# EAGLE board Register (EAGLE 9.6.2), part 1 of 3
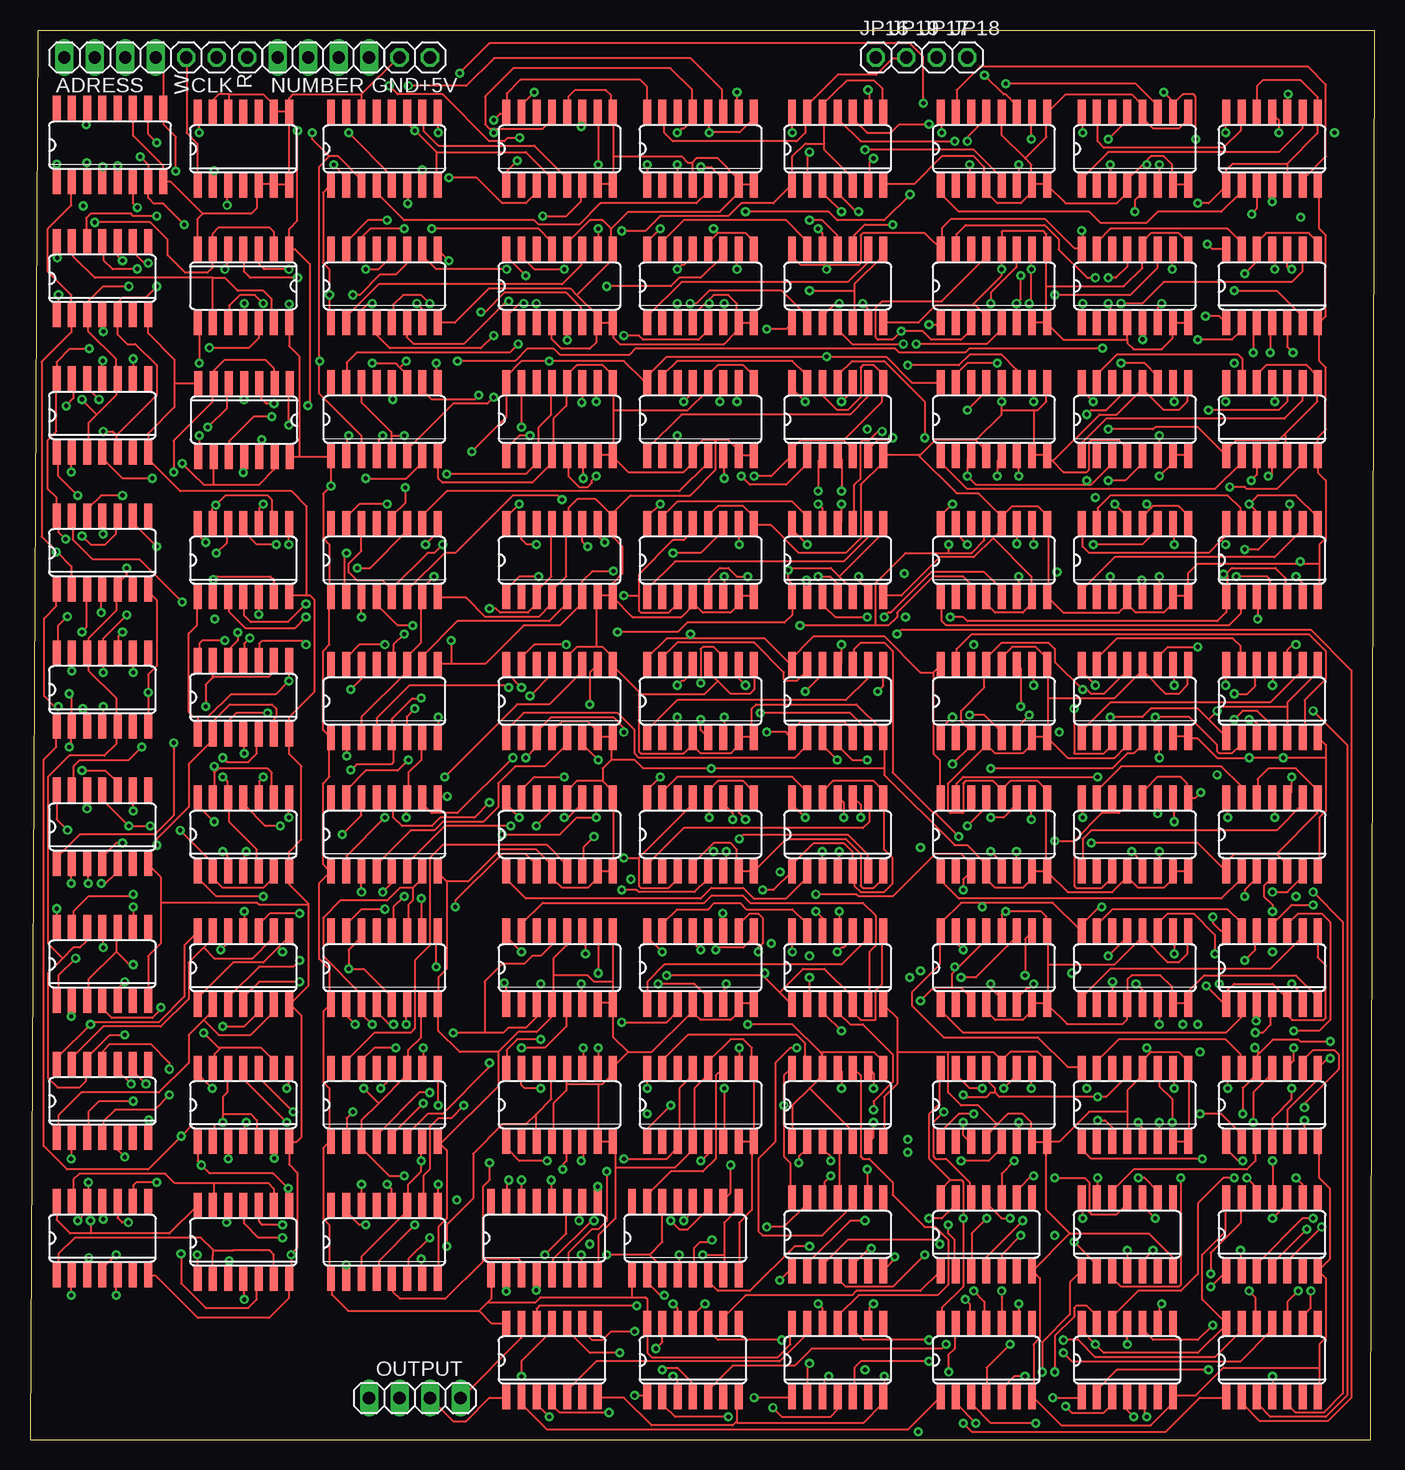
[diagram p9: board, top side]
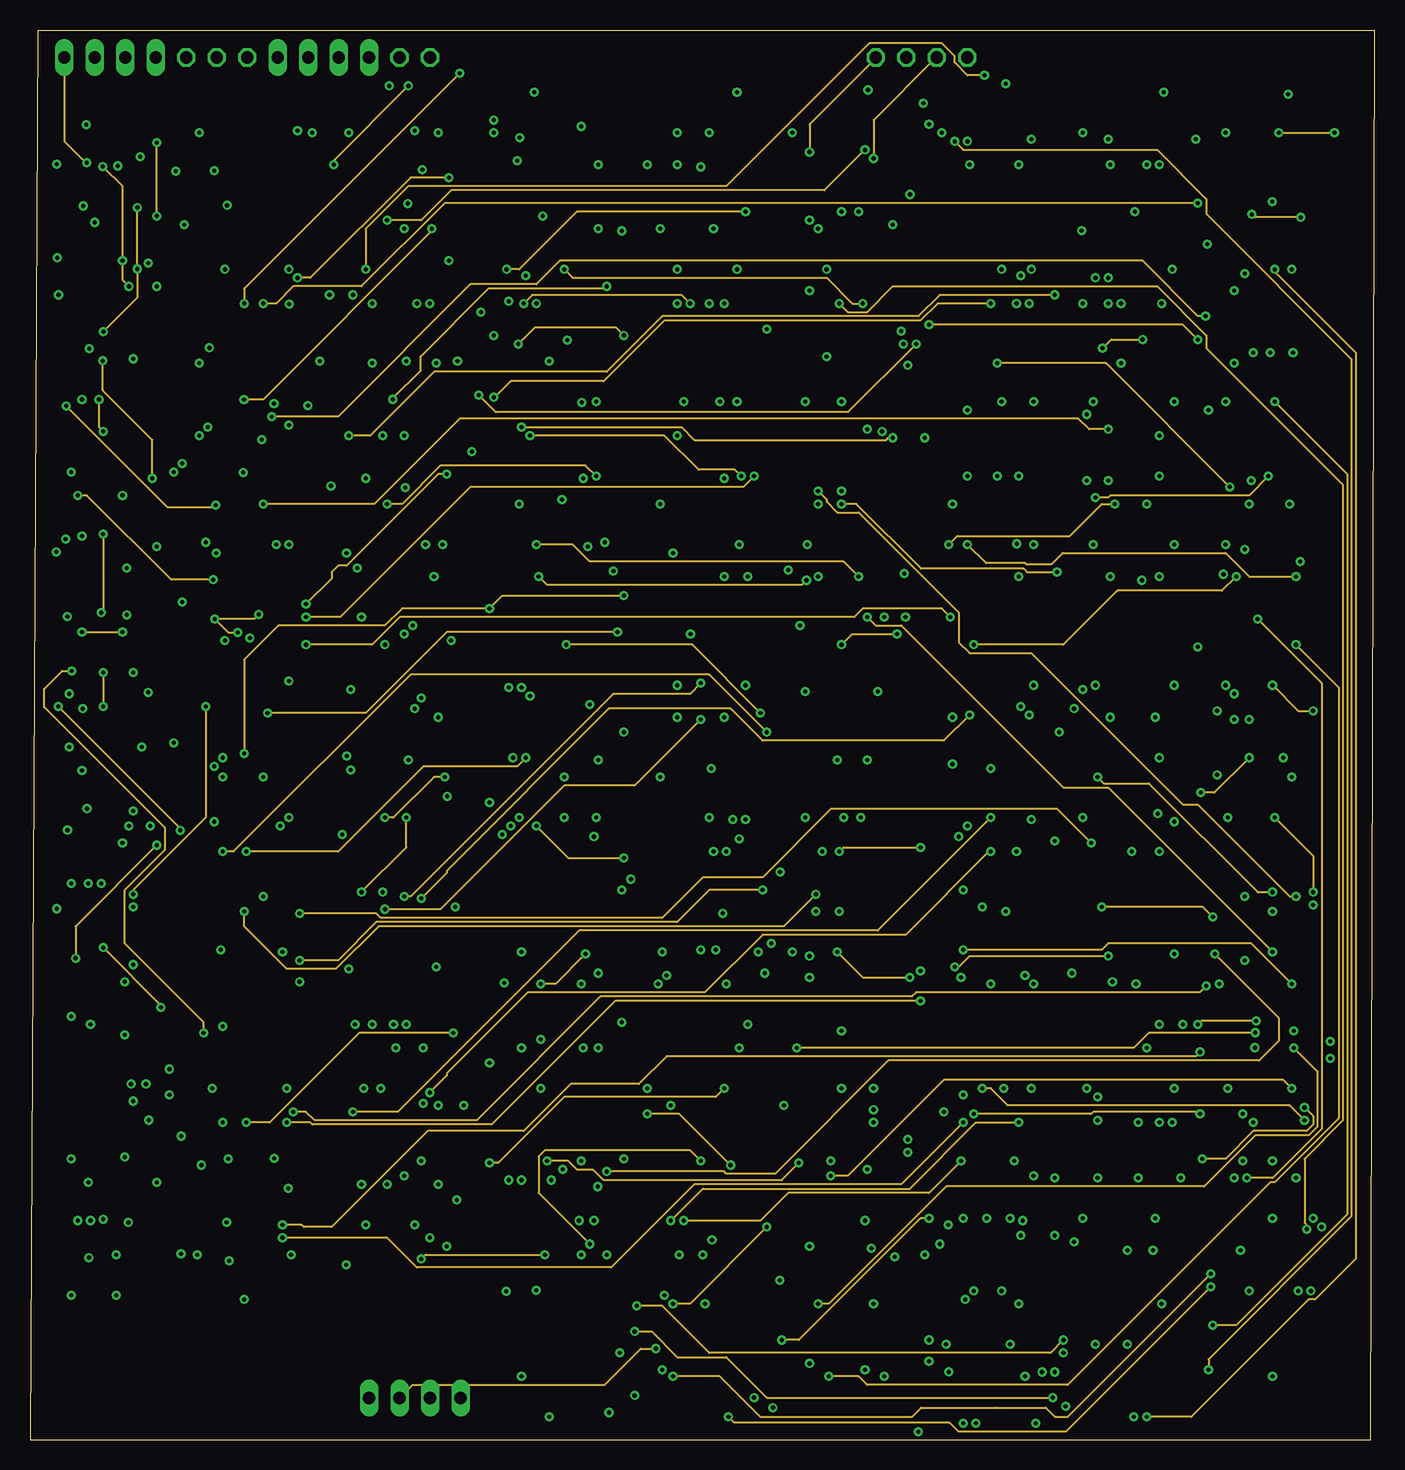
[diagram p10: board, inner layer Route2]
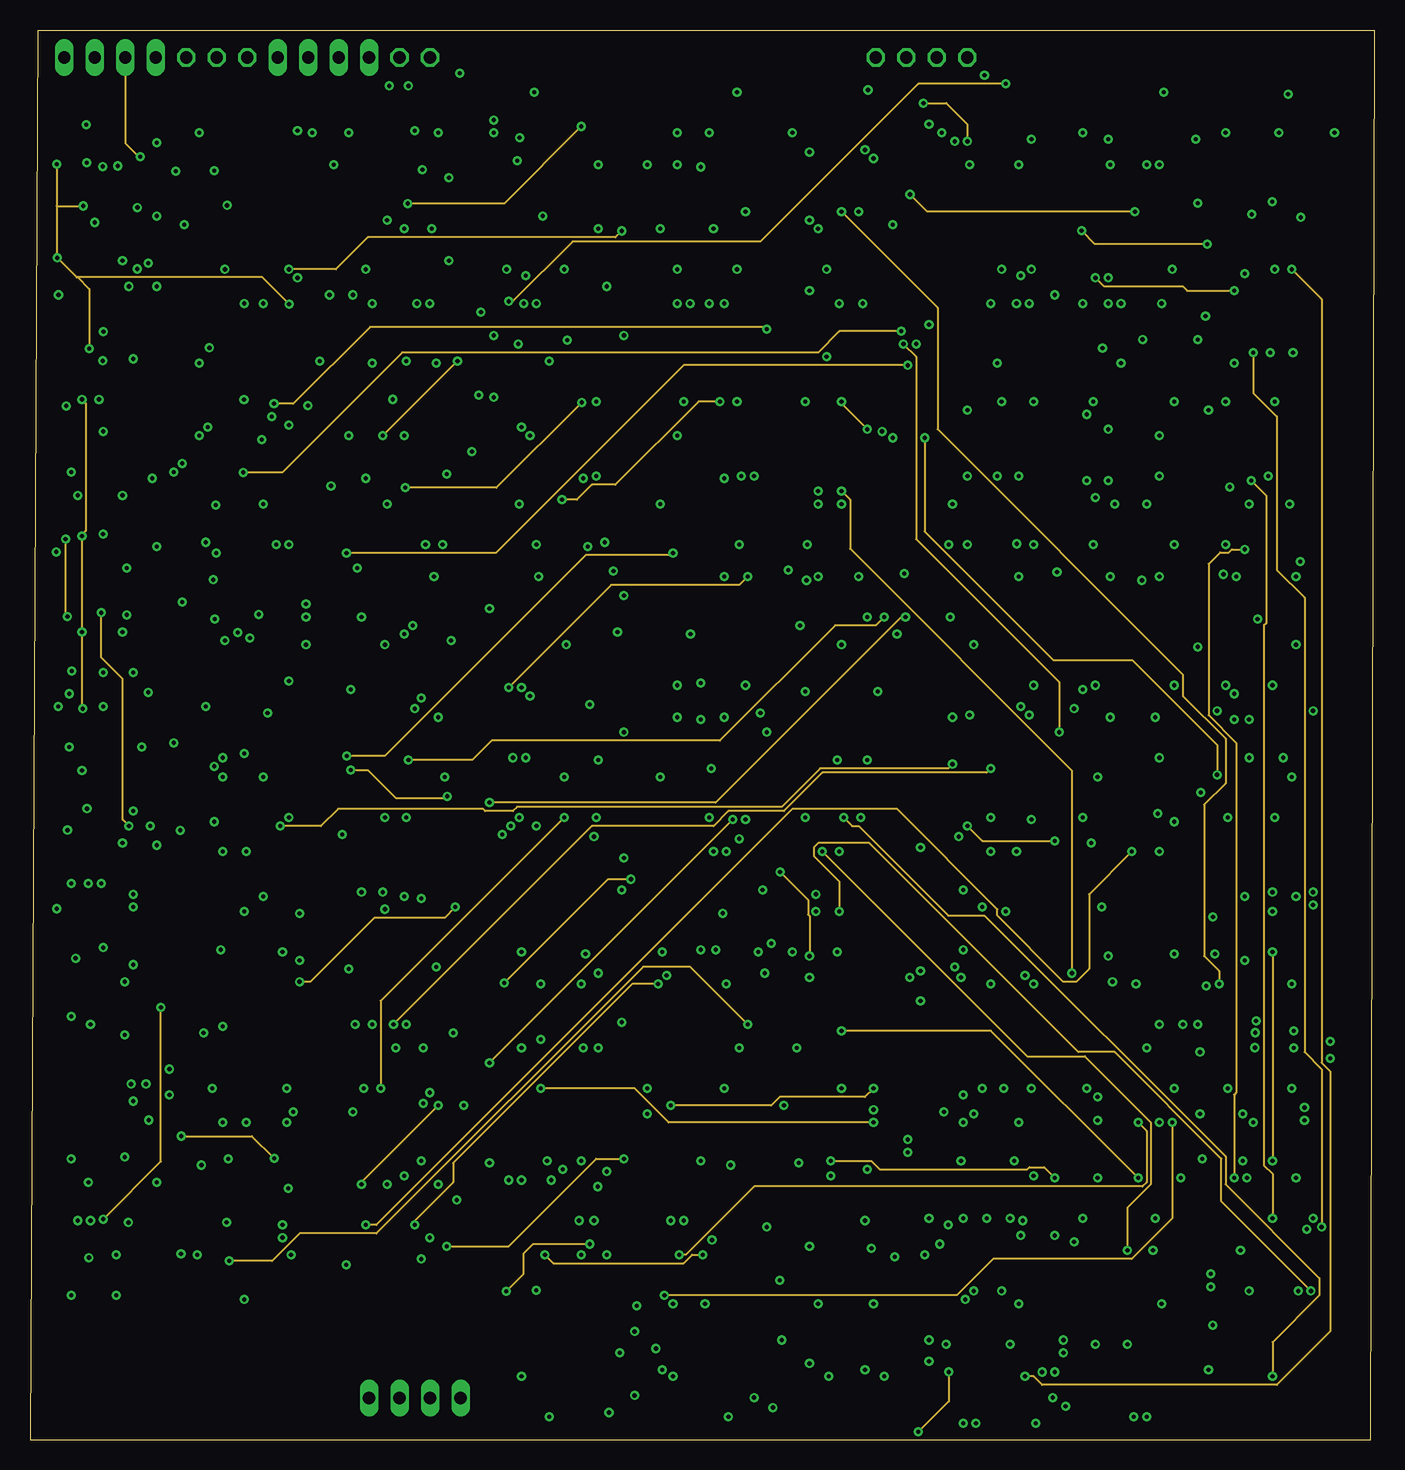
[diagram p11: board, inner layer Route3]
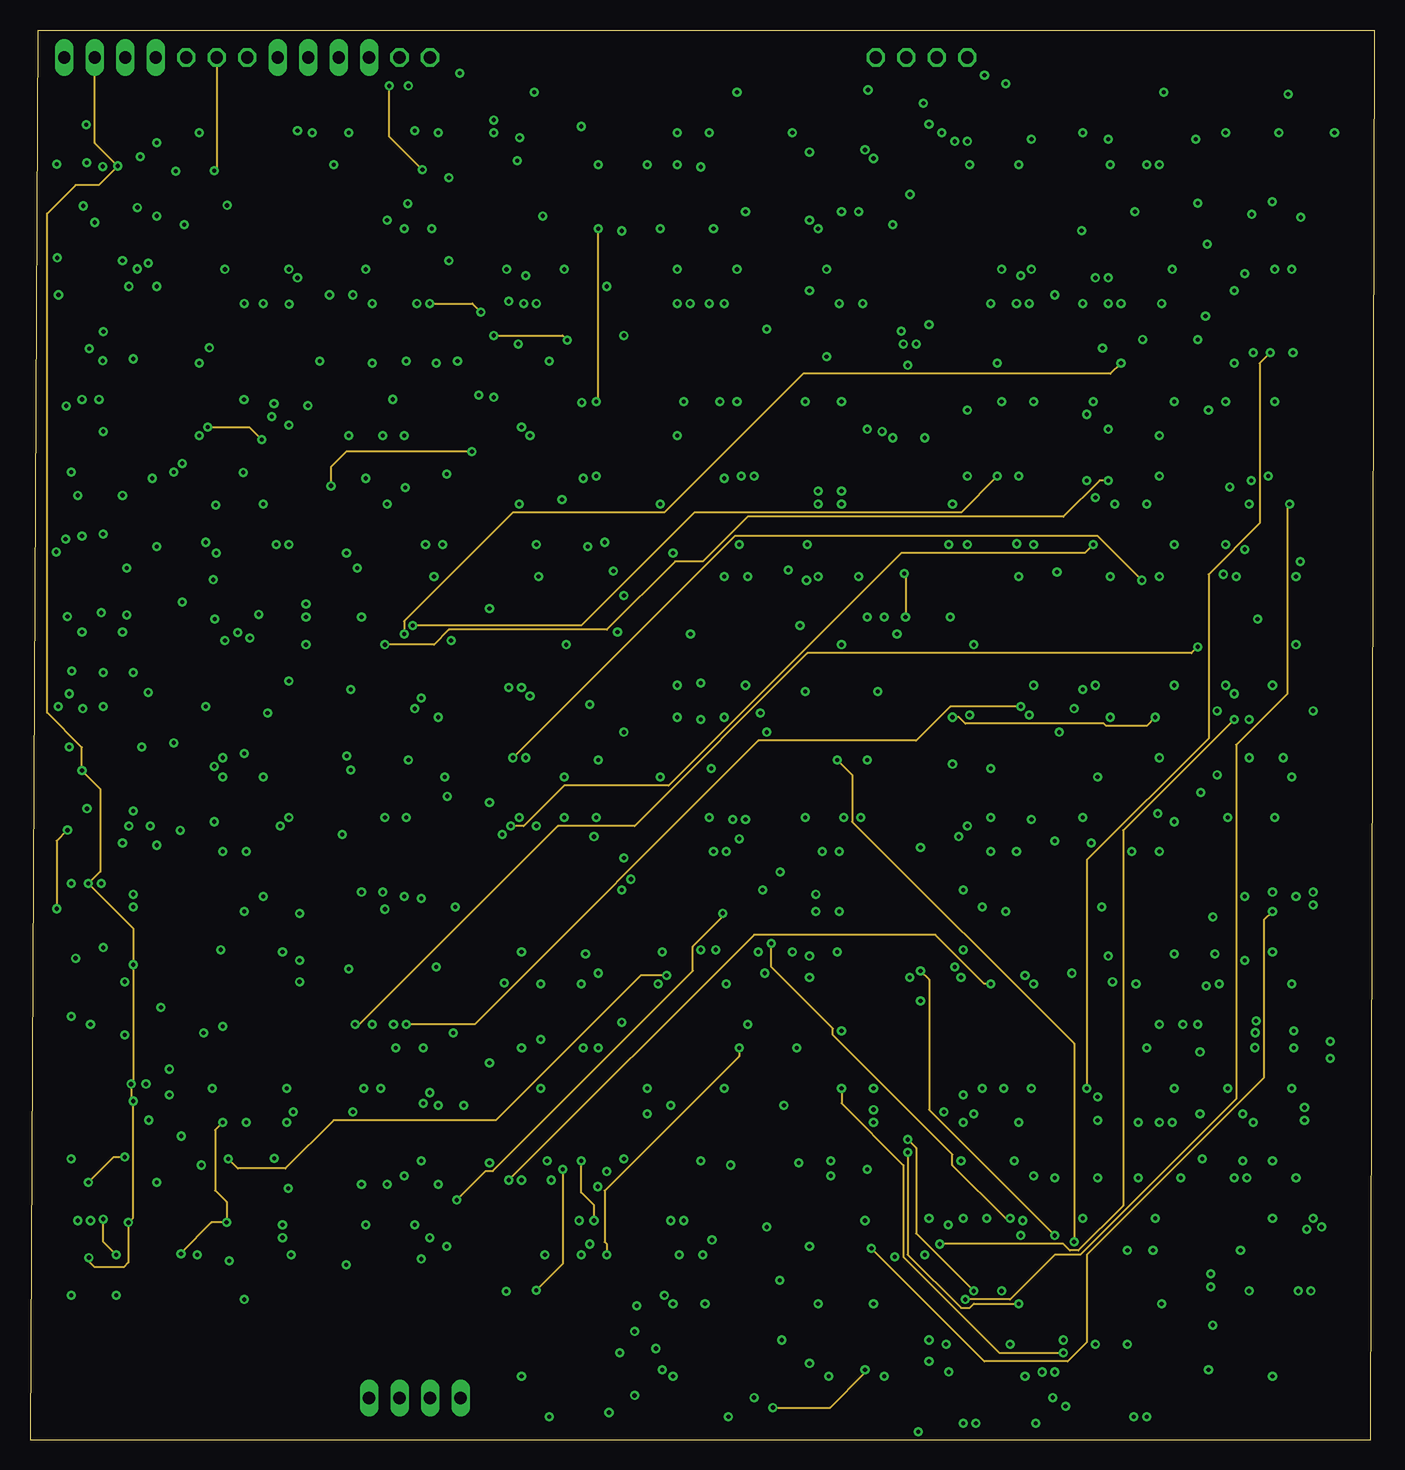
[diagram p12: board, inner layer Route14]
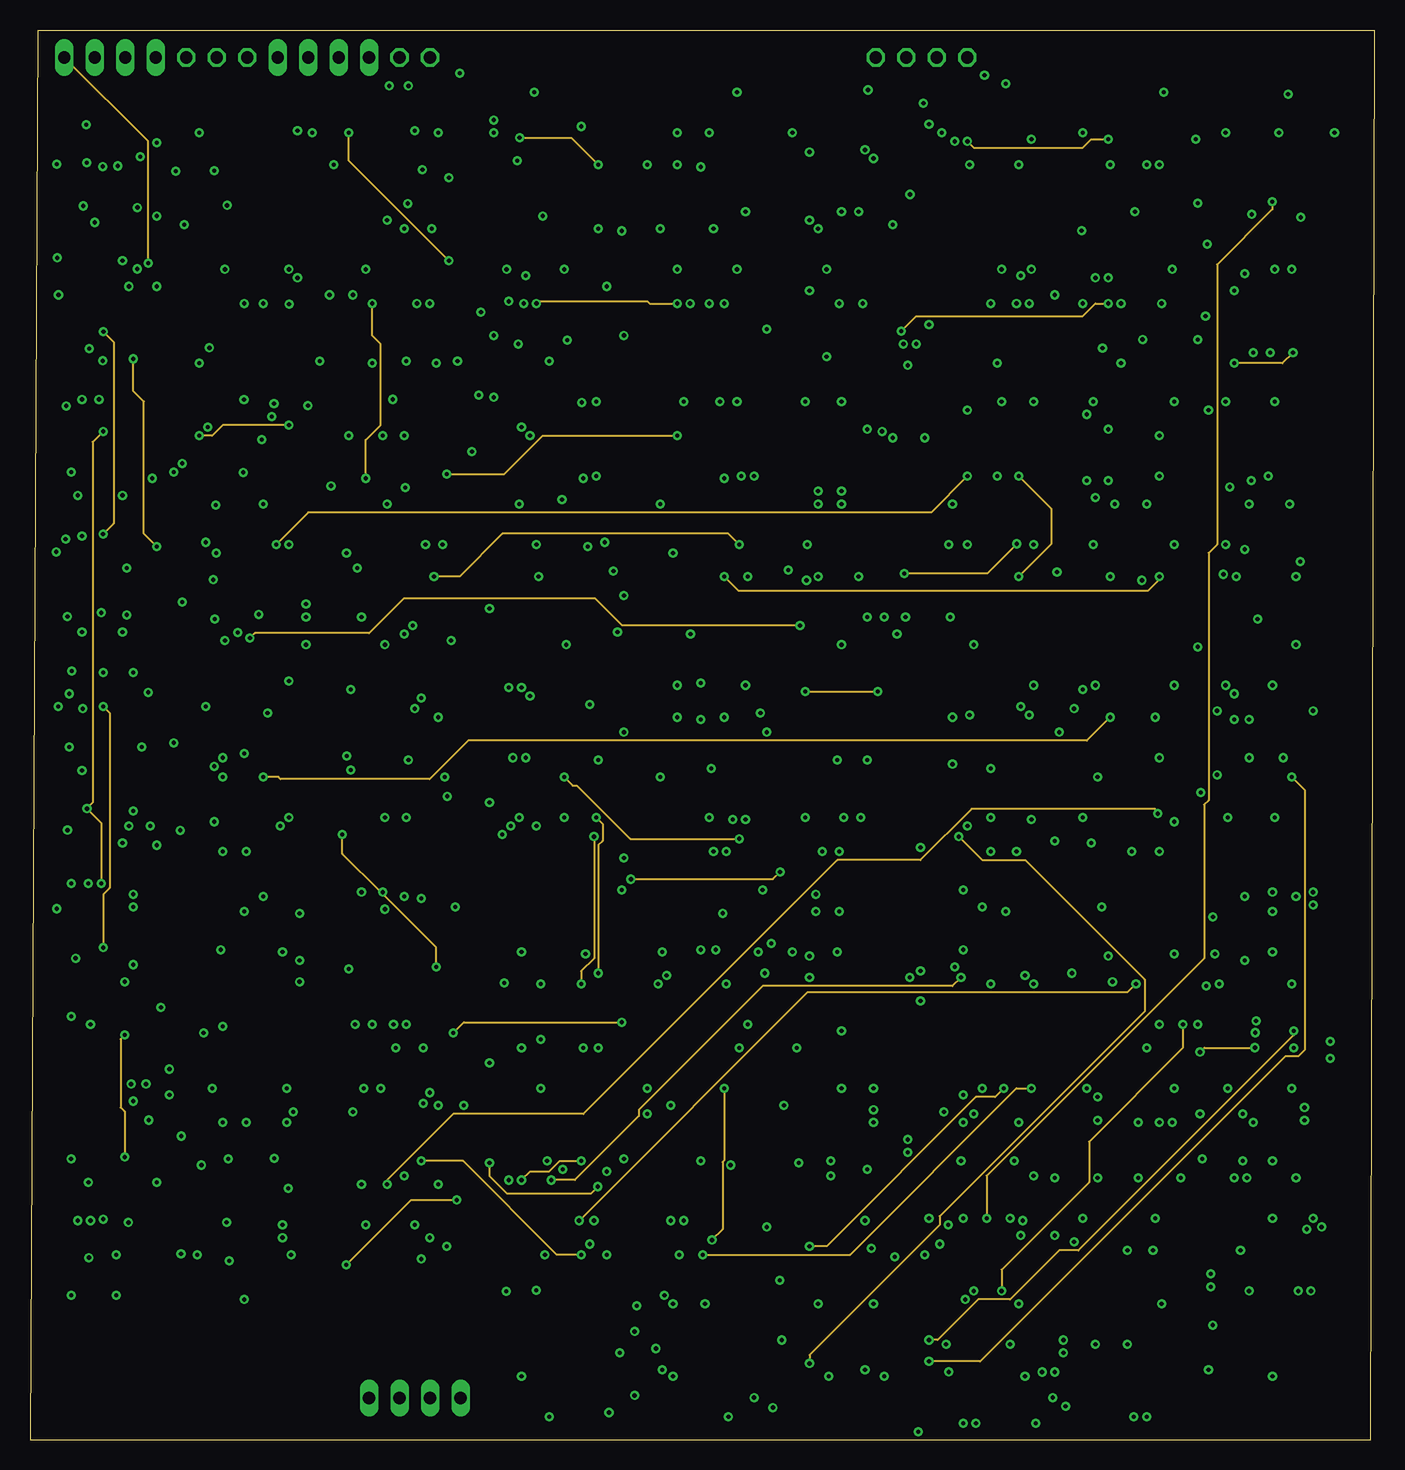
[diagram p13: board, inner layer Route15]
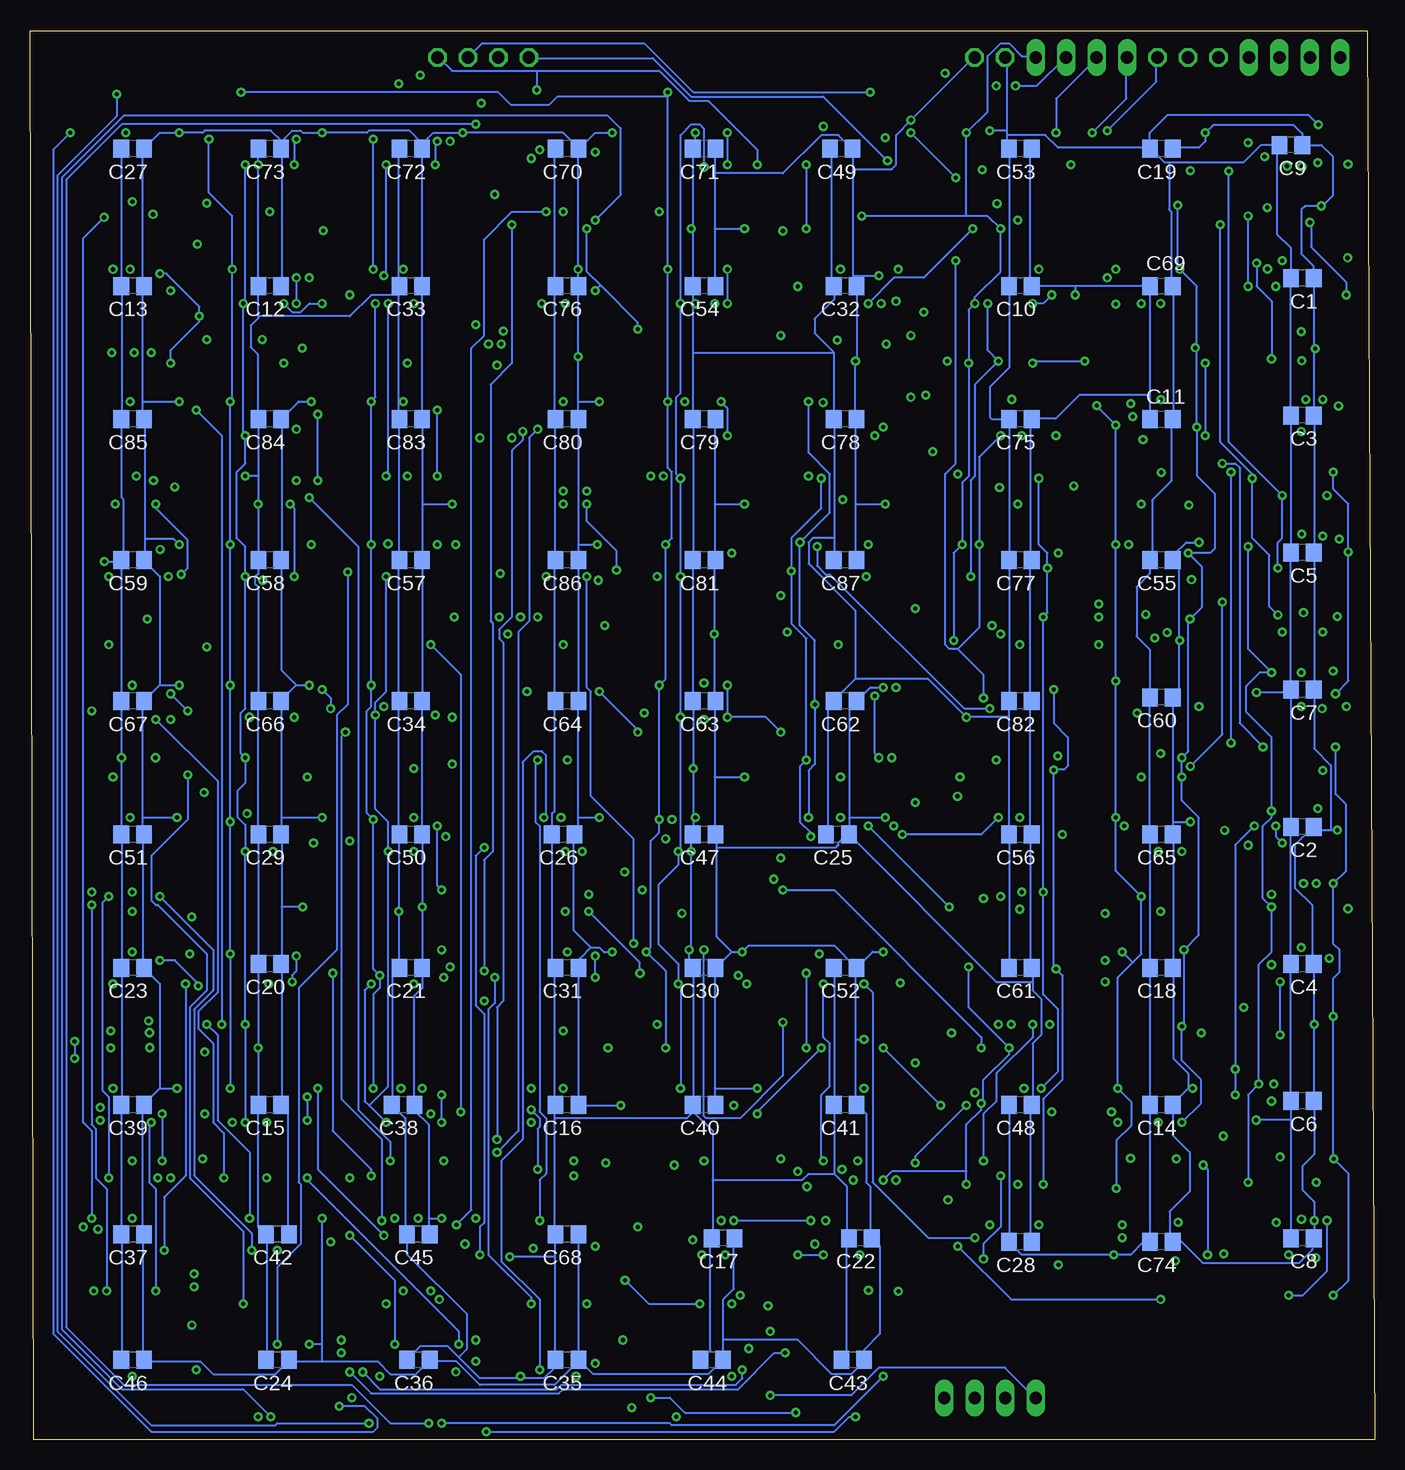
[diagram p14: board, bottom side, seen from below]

Size 112.06 x 117.46 mm. Coordinates in mm from the lower left corner, seen from the top.
Outline: 0,0 111.74,0 112.06,117.46 0.63,117.46 0,0
Copper layers (1+2*3+14*15+16): Top 0.035mm / dielectric 0.25mm / Route2 0.035mm / dielectric 0.25mm / Route3 0.035mm / dielectric 0.25mm / Route14 0.035mm / dielectric 0.25mm / Route15 0.035mm / dielectric 0.25mm / Bottom 0.035mm
Design rules "default *": minimum track width 6mil, minimum drill 0.35mm, track to track 8mil, track to pad 8mil, pad to pad 8mil, via to via 8mil, smd to smd 8mil, copper to edge 10mil, drill to drill 8mil, minimum pad ring 10mil, minimum via ring 8mil, stop-mask expansion 4mil, vias tented up to drill 0mil, thermal gap 10mil

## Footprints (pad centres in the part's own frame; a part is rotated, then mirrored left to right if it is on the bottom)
1X01 = drill 1.016 octagon: 1 0,0
1X04 = drill 1.016 long: 1 -3.81,0; 2 -1.27,0; 3 1.27,0; 4 3.81,0
C0805 = smd 1.3 x 1.5: 1 -0.95,0; 2 0.95,0
SO14 = smd 0.66 x 2.032: 1 -3.81,-3.073; 2 -2.54,-3.073; 3 -1.27,-3.073; 4 0,-3.073; 5 1.27,-3.073; 6 2.54,-3.073; 7 3.81,-3.073; 8 3.81,3.073; 9 2.54,3.073; 10 1.27,3.073; 11 0,3.073; 12 -1.27,3.073; 13 -2.54,3.073; 14 -3.81,3.073
SO16 = smd 0.66 x 2.032: 1 -4.445,-3.073; 2 -3.175,-3.073; 3 -1.905,-3.073; 4 -0.635,-3.073; 5 0.635,-3.073; 6 1.905,-3.073; 7 3.175,-3.073; 8 4.445,-3.073; 9 4.445,3.073; 10 3.175,3.073; 11 1.905,3.073; 12 0.635,3.073; 13 -0.635,3.073; 14 -1.905,3.073; 15 -3.175,3.073; 16 -4.445,3.073

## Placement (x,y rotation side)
+5V  [1X01]  33.34,115.25 0 top
ADRESS  [1X04]  6.67,115.25 0 top
C1  [C0805]  6.03,96.84 180 bottom
C2  [C0805]  6.03,51.12 180 bottom
C3  [C0805]  6.03,85.41 180 bottom
C4  [C0805]  6.03,39.69 180 bottom
C5  [C0805]  6.03,73.98 180 bottom
C6  [C0805]  6.03,28.26 180 bottom
C7  [C0805]  6.03,62.55 180 bottom
C8  [C0805]  6.03,16.83 180 bottom
C9  [C0805]  6.98,107.95 180 bottom
C10  [C0805]  29.53,96.2 180 bottom
C11  [C0805]  17.78,85.09 0 bottom
C12  [C0805]  92.08,96.2 180 bottom
C13  [C0805]  103.5,96.2 180 bottom
C14  [C0805]  17.78,27.94 180 bottom
C15  [C0805]  92.08,27.94 180 bottom
C16  [C0805]  67.31,27.94 180 bottom
C17  [C0805]  54.29,16.83 180 bottom
C18  [C0805]  17.78,39.37 180 bottom
C19  [C0805]  17.78,107.63 180 bottom
C20  [C0805]  92.08,39.69 180 bottom
C21  [C0805]  80.33,39.37 180 bottom
C22  [C0805]  42.86,16.83 180 bottom
C23  [C0805]  103.5,39.37 180 bottom
C24  [C0805]  91.44,6.67 180 bottom
C25  [C0805]  44.77,50.48 180 bottom
C26  [C0805]  67.63,50.48 180 bottom
C27  [C0805]  103.5,107.63 180 bottom
C28  [C0805]  29.53,16.51 180 bottom
C29  [C0805]  92.08,50.48 180 bottom
C30  [C0805]  55.88,39.37 180 bottom
C31  [C0805]  67.31,39.37 180 bottom
C32  [C0805]  44.13,96.2 180 bottom
C33  [C0805]  80.33,96.2 180 bottom
C34  [C0805]  80.33,61.59 180 bottom
C35  [C0805]  67.31,6.67 180 bottom
C36  [C0805]  79.69,6.67 180 bottom
C37  [C0805]  103.5,17.15 180 bottom
C38  [C0805]  80.96,27.94 180 bottom
C39  [C0805]  103.5,27.94 180 bottom
C40  [C0805]  55.88,27.94 180 bottom
C41  [C0805]  44.13,27.94 180 bottom
C42  [C0805]  91.44,17.15 180 bottom
C43  [C0805]  43.5,6.67 180 bottom
C44  [C0805]  55.24,6.67 180 bottom
C45  [C0805]  79.69,17.15 180 bottom
C46  [C0805]  103.5,6.67 180 bottom
C47  [C0805]  55.88,50.48 180 bottom
C48  [C0805]  29.53,27.94 180 bottom
C49  [C0805]  44.45,107.63 180 bottom
C50  [C0805]  80.33,50.48 180 bottom
C51  [C0805]  103.5,50.48 180 bottom
C52  [C0805]  44.13,39.37 180 bottom
C53  [C0805]  29.53,107.63 180 bottom
C54  [C0805]  55.88,96.2 180 bottom
C55  [C0805]  17.78,73.34 180 bottom
C56  [C0805]  29.53,50.48 180 bottom
C57  [C0805]  80.33,73.34 180 bottom
C58  [C0805]  92.08,73.34 180 bottom
C59  [C0805]  103.5,73.34 180 bottom
C60  [C0805]  17.78,61.91 180 bottom
C61  [C0805]  29.53,39.37 180 bottom
C62  [C0805]  44.13,61.59 180 bottom
C63  [C0805]  55.88,61.59 180 bottom
C64  [C0805]  67.31,61.59 180 bottom
C65  [C0805]  17.78,50.48 180 bottom
C66  [C0805]  92.08,61.59 180 bottom
C67  [C0805]  103.5,61.59 180 bottom
C68  [C0805]  67.31,17.15 180 bottom
C69  [C0805]  17.78,96.2 0 bottom
C70  [C0805]  67.31,107.63 180 bottom
C71  [C0805]  55.88,107.63 180 bottom
C72  [C0805]  80.33,107.63 180 bottom
C73  [C0805]  92.08,107.63 180 bottom
C74  [C0805]  17.78,16.51 180 bottom
C75  [C0805]  29.53,85.09 180 bottom
C76  [C0805]  67.31,96.2 180 bottom
C77  [C0805]  29.53,73.34 180 bottom
C78  [C0805]  44.13,85.09 180 bottom
C79  [C0805]  55.88,85.09 180 bottom
C80  [C0805]  67.31,85.09 180 bottom
C81  [C0805]  55.88,73.34 180 bottom
C82  [C0805]  29.53,61.59 180 bottom
C83  [C0805]  80.33,85.09 180 bottom
C84  [C0805]  92.08,85.09 180 bottom
C85  [C0805]  103.5,85.09 180 bottom
C86  [C0805]  67.31,73.34 180 bottom
C87  [C0805]  44.13,73.34 180 bottom
CLK  [1X01]  15.56,115.25 0 top
GND  [1X01]  30.8,115.25 0 top
IC1  4082D  [SO14]  6.03,96.84 0 top
IC2  4082D  [SO14]  6.03,51.12 0 top
IC3  4082D  [SO14]  6.03,85.41 0 top
IC4  4082D  [SO14]  6.03,39.69 0 top
IC5  4082D  [SO14]  6.03,73.98 0 top
IC6  4082D  [SO14]  6.03,28.26 0 top
IC7  4082D  [SO14]  6.03,62.55 0 top
IC8  4082D  [SO14]  6.03,16.83 0 top
IC9  4049D  [SO16]  6.67,107.95 0 top
IC10  4027D  [SO16]  44.13,107.63 0 top
IC11  4027D  [SO16]  55.88,107.63 0 top
IC12  4027D  [SO16]  80.33,107.63 0 top
IC13  4081D  [SO14]  17.78,73.34 0 top
IC14  4081D  [SO14]  67.31,107.63 0 top
IC15  4081D  [SO14]  17.78,96.2 180 top
IC16  4027D  [SO16]  92.08,107.63 0 top
IC17  4081D  [SO14]  17.78,61.91 0 top
IC18  4081D  [SO14]  103.5,107.63 0 top
IC19  4081D  [SO14]  17.84,85.03 180 top
IC20  4027D  [SO16]  44.13,96.2 0 top
IC21  4027D  [SO16]  55.88,96.2 0 top
IC22  4049D  [SO16]  54.61,16.83 0 top
IC23  4081D  [SO14]  67.31,96.2 0 top
IC24  4081D  [SO14]  17.78,50.48 0 top
IC25  4027D  [SO16]  80.33,96.2 0 top
IC26  4027D  [SO16]  92.08,96.2 0 top
IC27  4081D  [SO14]  17.78,39.37 0 top
IC28  4081D  [SO14]  103.5,96.2 0 top
IC29  4081D  [SO14]  17.78,27.94 0 top
IC30  4027D  [SO16]  44.13,85.09 0 top
IC31  4027D  [SO16]  55.88,85.09 0 top
IC32  4081D  [SO14]  17.78,16.51 0 top
IC33  4081D  [SO14]  67.31,85.09 0 top
IC34  4081D  [SO14]  17.78,107.63 0 top
IC35  4027D  [SO16]  80.33,85.09 0 top
IC36  4027D  [SO16]  92.08,85.09 0 top
IC38  4081D  [SO14]  103.5,85.09 0 top
IC40  4027D  [SO16]  44.13,73.34 0 top
IC41  4027D  [SO16]  55.88,73.34 0 top
IC43  4081D  [SO14]  67.31,73.34 0 top
IC45  4027D  [SO16]  80.33,73.34 0 top
IC46  4027D  [SO16]  92.08,73.34 0 top
IC48  4081D  [SO14]  103.5,73.34 0 top
IC50  4027D  [SO16]  44.13,61.59 0 top
IC51  4027D  [SO16]  55.88,61.59 0 top
IC53  4081D  [SO14]  67.31,61.59 0 top
IC55  4027D  [SO16]  80.33,61.59 0 top
IC56  4027D  [SO16]  92.08,61.59 0 top
IC58  4081D  [SO14]  103.5,61.59 0 top
IC60  4027D  [SO16]  44.13,50.48 0 top
IC61  4027D  [SO16]  55.88,50.48 0 top
IC63  4081D  [SO14]  67.31,50.48 0 top
IC65  4027D  [SO16]  80.33,50.48 0 top
IC66  4027D  [SO16]  92.08,50.48 0 top
IC68  4081D  [SO14]  103.5,50.48 0 top
IC70  4027D  [SO16]  44.13,39.37 0 top
IC71  4027D  [SO16]  55.88,39.37 0 top
IC73  4081D  [SO14]  67.31,39.37 0 top
IC75  4027D  [SO16]  80.33,39.37 0 top
IC76  4027D  [SO16]  92.08,39.37 0 top
IC78  4081D  [SO14]  103.5,39.37 0 top
IC80  4027D  [SO16]  44.13,27.94 0 top
IC81  4027D  [SO16]  55.88,27.94 0 top
IC83  4081D  [SO14]  67.31,27.94 0 top
IC85  4027D  [SO16]  80.33,27.94 0 top
IC86  4027D  [SO16]  92.08,27.94 0 top
IC88  4081D  [SO14]  103.5,27.94 0 top
IC90  4072D  [SO14]  103.5,17.15 0 top
IC91  4072D  [SO14]  91.44,17.15 0 top
IC92  4072D  [SO14]  55.24,6.67 0 top
IC93  4072D  [SO14]  79.69,17.15 0 top
IC94  4072D  [SO14]  67.31,17.15 0 top
IC96  4072D  [SO14]  79.69,6.67 0 top
IC97  4072D  [SO14]  67.31,6.67 0 top
IC98  4072D  [SO14]  43.5,6.67 0 top
IC99  4072D  [SO14]  91.44,6.67 0 top
IC100  4072D  [SO14]  103.5,6.67 0 top
IC108  4049D  [SO16]  42.86,16.83 0 top
IC109  4049D  [SO16]  29.53,16.51 0 top
IC110  4049D  [SO16]  29.53,27.94 0 top
IC111  4049D  [SO16]  29.53,39.37 0 top
IC112  4049D  [SO16]  29.53,50.48 0 top
IC113  4049D  [SO16]  29.53,61.59 0 top
IC114  4049D  [SO16]  29.53,73.34 0 top
IC115  4049D  [SO16]  29.53,85.09 0 top
IC116  4049D  [SO16]  29.53,96.2 0 top
IC117  4049D  [SO16]  29.53,107.63 0 top
JP16  [1X01]  70.48,115.25 0 top
JP17  [1X01]  75.56,115.25 0 top
JP18  [1X01]  78.11,115.25 0 top
JP19  [1X01]  73.03,115.25 0 top
NUMBER  [1X04]  24.45,115.25 180 top
OUTPUT  [1X04]  32.07,3.49 0 top
R  [1X01]  18.1,115.25 0 top
W  [1X01]  13.02,115.25 0 top

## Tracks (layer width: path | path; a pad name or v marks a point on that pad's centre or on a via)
0000  (via drill 0.35)
  Top 0.152: v2.37,95.45 2.37,93.85 IC1.1 | v5.4,101.5 10.02,101.5 11.47,100.04 11.47,98.76 12.92,97.31 14.78,97.31 15.18,97.7 15.18,99.19 IC15.6 15.2,99.32 15.2,100.53 15.75,101.09 19.94,101.09 20.31,100.71 IC15.2
  Bottom 0.152: v2.37,95.45 2.37,96.52 5.29,99.44 5.29,101.39 v5.4,101.5
0001
  Top 0.152: IC15.13 20.15,93.14 20.15,95.1 19.44,95.81 17.31,95.81 16.24,96.88 15.24,96.88 | 15.24,96.88 5.4,96.88 3.62,98.65 3.62,99.9 IC1.13 | IC15.9 15.24,96.88
0010  (via drill 0.35)
  Top 0.152: v11.98,58.11 11.98,52.07 10.38,50.47 4.15,50.47 2.37,48.69 2.37,48.16 IC2.1 | v11.98,80.7 11.98,83.3 15.18,86.5 15.18,87.99 IC19.6 15.35,88.16 15.35,89.17 16.22,90.04 19.62,90.04 20.33,89.33 20.33,88.16 IC19.2
  Bottom 0.152: v11.98,80.7 v11.98,58.11
0011  (via drill 0.35)
  Top 0.152: v9.31,57.76 8.2,56.65 4.11,56.65 3.62,56.16 3.62,54.2 IC2.13 | v12.69,81.41 13.58,80.52 14.47,79.63 15.4,79.63 | IC19.9 15.18,81.94 15.18,81.23 IC19.9 | IC19.13 20.33,81.94 20.33,80.87 19.09,79.63 16.78,79.63 15.4,79.63 | 15.4,79.63 15.3,79.72 IC19.9
  Bottom 0.152: v9.31,57.76 9.31,57.8 11.26,59.76 11.26,81.05 11.62,81.41 v12.69,81.41
0100  (via drill 0.35)
  Top 0.152: v3.98,78.74 2.37,80.34 2.37,82.3 IC3.1 | IC13.6 20.31,71.71 20.04,71.98 15.54,71.98 v15.27,71.71 15.24,71.69 IC13.2
  Route2 0.152: v3.98,78.74 4.74,78.74 11.77,71.71 v15.27,71.71
0101  (via drill 0.35)
  Top 0.152: 15.18,76.96 15.18,76.43 IC13.13 15.18,76.96 | IC3.13 3.62,88.34 3.62,86.84 3.02,86.23 v3.02,86.2 | IC13.9 20.15,76.43 20.15,78.38 19.8,78.74 16.95,78.74 16.27,78.74 v15.48,77.95 15.16,77.63 15.16,76.95 15.18,76.96
  Route2 0.152: v3.02,86.2 11.43,77.79 15.32,77.79 v15.48,77.95
0110  (via drill 0.35)
  Top 0.152: v3.8,40.16 2.37,38.73 2.37,36.78 IC4.1 | v10.55,49.58 10.55,50.11 13.22,52.78 13.22,56.34 15.18,58.29 15.18,58.83 IC17.2 15.35,59 15.35,60.01 16.66,61.32 20.15,61.32 20.51,60.96 20.51,60.25 20.33,60.07 20.33,59 IC17.6
  Route2 0.152: v3.8,40.16 3.8,42.82 v10.55,49.58
0111  (via drill 0.35)
  Top 0.152: v8.6,45.49 8.42,45.31 4.86,45.31 3.62,44.07 3.62,42.82 IC4.13 | v14.64,61.14 14.64,62.96 15.24,63.56 15.24,63.66 | 15.24,63.66 IC17.13 | IC17.9 20.15,64.87 20.15,63.86 19.95,63.66 15.24,63.66
  Route2 0.152: v8.6,45.49 8.6,45.85 14.64,51.89 v14.64,61.14
1000  (via drill 0.35)
  Top 0.152: IC24.6 20.15,47.27 20.15,46.74 19.44,46.03 16.07,46.03 15.35,46.74 15.35,47.27 IC24.2 15.18,47.45 15.18,48.16 v12.51,50.83 | v2.36,61.14 2.04,61.14 1.17,62.01 1.17,68.49 2.2,69.52 2.2,70.74 IC5.1
  Route2 0.152: v12.51,50.83 12.51,50.98 v2.36,61.14
1001  (via drill 0.35)
  Top 0.152: 15.35,55.63 15.35,53.67 IC24.13 | 15.35,55.63 15.71,55.98 19.8,55.98 20.15,55.63 20.15,53.67 IC24.9 | v12.69,69.85 9.13,73.41 5.22,73.41 3.62,75.01 3.62,76.96 IC5.13 | 15.35,55.63 v15.35,56.16
  Bottom 0.152: v12.69,69.85 12.69,58.83 v15.35,56.16
1010
  Top 0.152: 14.47,35 15.18,35.71 15.18,36.25 IC27.2 | 14.47,35 13.22,33.76 13.22,31.45 10.73,28.96 4.29,28.96 2.37,27.05 2.37,25.22 IC6.1 | 14.47,35 15.71,33.76 18.38,33.76 20.15,35.53 20.15,36.25 IC27.6
1011
  Top 0.152: 14.47,41.05 15.18,41.76 15.18,42.29 IC27.13 | 14.47,41.05 13.22,39.8 13.22,36.78 10.91,34.47 6.11,34.47 3.62,31.98 3.62,31.45 IC6.13 | 14.47,41.05 15.35,40.16 18.55,40.16 20.15,41.76 20.15,42.29 IC27.9
1100  (via drill 0.35)
  Top 0.152: IC29.2 15.35,24.87 15.35,26.29 13.58,26.29 v12.61,25.33 9.84,22.55 3.09,22.55 1.13,24.51 1.13,56.72 2.2,57.78 2.2,59.36 IC7.1 | v20.35,23.47 20.32,23.5 IC29.6
  Route3 0.152: v12.61,25.33 18.49,25.33 v20.35,23.47
1101  (via drill 0.35)
  Top 0.152: 15.89,32.69 15.35,32.16 15.35,31.09 IC29.13 | 15.89,32.69 19.27,32.69 20.15,31.8 20.15,31.09 IC29.9 | v3.47,64.11 3.44,64.14 3.44,65.58 IC7.13 | v14.47,33.93 15.71,32.69 15.89,32.69
  Route2 0.152: v3.47,64.11 2.67,64.11 1.17,62.61 1.17,61.1 11.26,51 11.26,49.23 7.89,45.85 7.89,41.4 14.47,34.82 v14.47,33.93
1110
  Top 0.152: IC32.6 20.33,13.49 20.33,15.44 19.98,15.8 19.37,15.8 16.95,15.8 15.32,15.8 15.24,15.88 | IC8.1 2.37,13.84 2.37,15.51 3.73,16.87 14.25,16.87 15.24,15.88 | IC32.2 15.24,15.38 15.24,15.88
1111
  Top 0.152: 15.35,21.43 15.35,19.71 IC32.13 | IC32.9 20.27,19.62 20.32,19.67 20.32,20.96 19.84,21.43 15.35,21.43 | IC8.13 3.62,20.07 3.62,21.71 4.11,22.2 11.27,22.2 12.04,21.43 15.35,21.43
+5V  (via drill 0.35)
  Top 0.152: v15.18,29.31 14.11,30.38 14.11,30.91 IC29.14 | v15.35,51.54 14.11,52.78 14.11,53.49 IC24.14 | v16.24,66.65 14.36,66.65 14.11,66.4 14.11,65.05 IC17.14 | v14.64,74.83 14.11,75.36 14.11,76.25 IC13.14 | v2.96,75.1 2.37,75.69 2.37,76.96 IC5.14 2.22,78.54 1.49,79.28 1.49,83.36 2.2,84.07 2.2,88.34 IC3.14 2.22,89.87 3.31,90.96 v4.95,90.96 | IC7.14 2.37,65.76 2.37,67.89 v3.12,68.64 | IC1.14 2.24,99.91 2.26,99.89 v2.26,98.54 | IC6.14 2.37,31.45 2.37,31.98 v5.04,34.65 5.22,34.82 10.73,34.82 12.87,36.96 12.87,41.22 13.93,42.29 IC27.14 | IC8.14 2.22,18.35 3.34,17.22 5.04,17.22 | 5.04,17.22 11.62,17.22 13.93,19.53 IC32.14 | v5.04,18.29 5.04,17.22 | IC2.14 2.22,51.75 v3.12,50.84 | v14.11,108.97 14.11,110.57 IC34.14 | v52.51,100.97 51.45,99.9 51.45,99.37 IC21.16 | IC11.16 51.44,112.8 50.86,113.37 40.86,113.37 39.71,112.23 39.71,110.74 IC10.16 39.54,110.57 39.18,110.57 v38.65,110.03 | v40.78,78.03 39.71,76.96 39.71,76.43 IC40.16 | v41.31,97.05 39.71,98.65 39.71,99.19 IC20.16 | 51.09,88.34 51.27,88.16 IC31.16 | 51.09,88.34 49.49,89.94 v43.27,89.94 40.96,89.94 39.71,88.7 39.71,88.16 IC30.16 39.69,85.25 v36.83,82.39 | IC35.16 73.49,88.16 71.36,90.3 v66.38,90.3 53.05,90.3 51.09,88.34 | 37.42,10.76 38.44,9.74 IC98.14 | IC108.1 38.47,13.67 38.47,11.81 38.15,11.49 | IC97.14 63.36,9.58 63.36,7.98 62.29,6.91 51.8,6.91 51.45,7.26 51.45,9.58 IC92.14 51.43,11.75 51.28,11.91 50.16,11.91 | 22.45,81.94 25.01,81.94 IC115.1 v25.08,79.53 | 22.45,81.94 21.76,81.94 IC19.14 | 22.45,81.94 22.45,90.34 21.59,91.2 IC15.14 21.58,93.14 21.58,94.68 v21.59,94.69 | 24.96,24.87 24.42,24.33 24.42,18.47 24.96,17.93 24.96,13.49 IC109.1 25.13,13.31 25.13,12.14 26.52,10.76 37.42,10.76
  Top 0.152: 24.96,24.87 24.96,29.31 24.42,29.85 24.42,35.71 24.96,36.25 IC111.1 24.96,36.42 24.96,39.27 24.07,40.16 24.07,46.38 24.96,47.27 IC112.1 24.96,47.45 24.42,47.98 24.42,54.74 24.96,55.27 24.96,58.47 IC113.1 24.42,59.18 24.42,65.76 24.96,66.29 24.96,70.21 IC114.1 24.96,70.38 24.96,74.65 24.42,75.18 24.42,78.87 25,79.45 | 24.96,24.87 IC110.1 | v88.61,86.56 87.72,87.45 87.72,88.16 IC36.16 | v87.72,51.89 87.72,53.49 IC66.16 | v88.79,62.92 87.72,63.98 87.72,64.52 IC56.16 | 79.36,44.78 85.23,44.78 87.34,42.67 | 79.36,44.78 77.58,44.78 75.98,43.18 75.98,42.47 IC75.16 75.81,42.29 75.81,39.62 73.49,37.31 73.49,36.25 76.16,33.58 83.99,33.58 86.47,31.09 87.54,31.09 IC86.16 | 87.34,42.67 87.54,42.47 IC76.16 | 87.34,42.67 89.12,44.44 89.32,44.44 v89.32,44.42 | 99.81,42.29 IC78.14 99.22,42.44 98.58,43.08 98.58,43.66 98.58,43.65 v98.58,43.59 | 76.7,21.67 77.58,21.67 77.76,21.49 v77.76,18.47 77.76,12.78 75.98,11 75.98,9.75 IC96.14 | 76.7,21.67 75.98,20.96 75.98,20.24 IC93.14 | 76.7,21.67 74.92,23.44 74.92,27.18 75.81,28.07 75.81,30.91 IC85.16 | v79.36,44.42 79.36,44.78 | IC99.14 87.72,9.58 87.72,9.04 v88.79,7.98 89.5,7.26 97.32,7.26 99.63,9.58 IC100.14 99.63,9.75 97.68,11.71 97.68,15.44 99.63,17.4 99.63,20.07 IC90.14 | v87.72,18.47 87.72,20.07 IC91.14 | v99.81,29.31 99.81,30.91 IC88.14 | v99.81,51.89 99.81,53.49 IC68.14 | v99.63,62.92 99.63,64.52 IC58.14 | 99.28,75.01 99.63,75.36 99.63,76.25 IC48.14 | 99.28,75.01 98.21,73.94 88.25,73.94 87.72,74.47 87.72,76.25 IC46.16 | v99.63,86.56 99.63,88.16 IC38.14 | v99.63,108.97 99.63,110.57 IC18.14 | v99.63,74.65 99.28,75.01
  Top 0.152: v87.72,108.97 87.72,110.57 IC16.16 | v76.87,78.03 75.98,77.14 75.98,76.43 IC45.16 | v75.98,108.97 75.98,110.57 IC12.16 | v64.6,51.89 63.54,52.96 63.54,53.49 IC63.14 | IC94.14 63.36,20.24 63.36,23.09 62.83,23.62 v62.83,27.89 62.83,30.38 63.36,30.91 IC83.14 | v63.54,40.69 63.54,42.29 IC73.14 | 66.38,97.94 69.05,97.94 69.23,98.12 69.23,100.43 69.41,100.61 74.56,100.61 75.07,100.1 75.63,99.54 | 66.38,97.94 64.25,97.94 63.54,98.65 63.54,99.19 IC23.14 | 75.68,99.49 75.81,99.37 IC25.16 75.63,99.54 | 75.68,99.49 75.63,99.54 | v64.78,74.65 63.54,75.89 63.54,76.25 IC43.14 | v64.6,86.56 63.54,87.63 63.54,88.16 IC33.14 | v63.54,108.97 63.54,110.57 IC14.14 | v66.38,97.59 66.38,97.94 | IC116.1 24.96,93.14 v24.96,95.45 24.96,97.59 24.42,98.12 24.42,103.99 24.96,104.52 IC117.1 | v42.56,33.4 40.6,33.4 39.71,32.51 39.71,31.09 IC80.16 | v40.96,40.69 39.71,41.94 39.71,42.29 IC70.16 | 75.27,63.98 75.27,57.23 75.81,56.69 75.81,53.67 IC65.16 | 75.27,63.98 75.81,64.52 IC55.16 | 55.04,66.83 61.23,66.83 63.18,64.87 | 55.04,66.83 53.05,66.83 51.45,65.23 51.45,64.69 IC51.16 | 63.18,64.87 63.36,64.69 IC53.14 63.18,64.87 | 75.27,63.98 74.21,63.98 71.18,67 65.32,67 63.18,64.87 | v40.78,51.89 39.71,52.96 39.71,53.49 IC60.16 | v40.96,62.74 39.71,63.98 39.71,64.52 IC50.16 | v52.51,78.03 51.45,76.96 51.45,76.43 IC41.16 | v52.51,55.27 51.45,54.2 51.45,53.67 IC61.16 | v51.45,29.31 51.45,30.91 IC81.16 | v52.69,40.69 51.45,41.94 51.45,42.29 IC71.16 | v55.04,67.18 55.04,66.83 | IC9.1 v2.22,106.36 | v2.22,44.29 IC4.14 | v25.08,79.53 25.08,79.45 25.01,79.45 25,79.45 | v25.08,79.53 25,79.45 | 37.42,10.76 38.15,11.49 | 50.16,11.91 42.55,11.91 42.13,11.49 38.15,11.49
  Top 0.152: IC22.1 50.16,11.91 | IC28.14 98.53,99.28 v98.11,99.7 | v87.63,100.81 87.72,100.72 87.72,99.37 IC26.16 87.54,99.37 87.01,99.37 84.58,101.8 76.77,101.8 75.99,101.02 75.99,99.8 75.68,99.49
  Route2 0.152: v98.58,43.59 97.74,44.42 v89.32,44.42
  Route3 0.152: v2.22,106.36 2.22,102.87 | 2.22,102.87 2.22,98.9 2.26,98.86 v2.26,98.54 3.89,96.91 3.97,96.91 | v21.59,94.69 19.37,96.91 3.97,96.91 | 3.97,96.91 4.95,95.94 v4.95,90.96 | 2.22,102.87 v4.45,102.87 | v3.12,68.64 2.96,68.79 v2.96,75.1 | v98.11,99.7 88.74,99.7 v87.63,100.81
  Route14 0.152: v3.12,50.84 2.22,49.94 v2.22,44.29 | v36.83,82.39 26.35,82.39 25.08,81.12 v25.08,79.53
  Bottom 0.152: 15.53,29.31 16.78,28.07 C14.1 16.83,25.4 15.4,23.97 15.4,20.75 17.09,19.05 17.09,16.51 C74.1 16.07,16.51 14.29,14.73 6.34,14.73 5.22,15.86 5.22,16.69 C8.1 5.04,16.87 v5.04,18.29 5.04,19.84 6.03,20.83 6.03,22.82 5.04,23.81 5.04,28.25 C6.1 5.04,28.42 v5.04,34.65 5.04,39.62 C4.1 5.22,39.8 5.22,44.6 6.64,46.03 6.64,49.58 5.22,51 C2.1 5.04,51.18 5.04,50.84 3.65,50.84 | 16.78,51.54 16.78,50.65 C65.1 16.78,50.47 16.78,39.45 C18.1 16.78,39.27 16.78,31.8 15.53,30.56 15.53,29.31 | 16.78,51.54 16.78,61.85 C60.1 16.3,62.44 16.3,66.71 | 16.3,66.71 16.3,72.81 C55.1 16.78,73.41 16.78,73.76 15.71,74.83 v14.64,74.83 | 16.78,51.54 v15.35,51.54 | 16.3,66.71 v16.24,66.65 | 15.53,29.31 v15.18,29.31 | 3.65,50.84 v3.12,50.84 | C19.1 16.78,107.72 14.66,107.72 14.11,108.27 v14.11,108.97 13.46,109.62 6.75,109.62 6.04,108.9 C9.1 4.45,107.95 3.49,107 3.49,103.74 4.36,102.87 v4.45,102.87 5.79,102.87 6.11,102.55 6.11,98.88 5.08,97.85 C1.1 5.04,96.7 5.04,90.96 | 5.04,90.96 5.04,85.5 C3.1 5.04,85.32 5.04,74.12 C5.1 5.04,73.94 5.04,62.56 C7.1 5.04,62.38 5.04,57.63 3.65,56.24 3.65,50.84 | 5.04,90.96 v4.95,90.96 | 55,105.59 55,107.54 C71.1 | 55,105.59 55,100.97 | 55,100.97 55,96.34 C54.1 | 55,100.97 v52.51,100.97 | 43.27,78.03 43.27,84.96 C78.1 43.27,85.14 v43.27,89.94 43.27,90.01 43.18,90.1 C32.1 43.27,96.34 43.45,96.52 43.45,97.05 | 43.27,78.03 43.27,73.41 C87.1 | 43.45,97.05 43.45,105.94 | 43.45,105.94 43.45,107.54 C49.1 43.62,107.72 44.69,108.79 46.11,108.79 49.31,105.59 55,105.59 | 43.27,78.03 v40.78,78.03 | 43.45,97.05 v41.31,97.05 | 43.45,105.94 40.25,105.94 39.89,106.3 39.89,108.79 v38.65,110.03 33.49,115.19 +5V.1
  Bottom 0.152: v88.61,86.56 89.67,86.56 91.1,85.14 C84.1 91.1,84.96 91.1,73.41 C58.1 91.1,73.23 91.1,64.16 89.85,62.92 | C42.1 90.56,17.22 90.56,27.36 91.1,27.89 C15.1 91.1,28.07 91.1,39.62 C20.1 91.1,39.8 91.1,44.42 | 91.1,44.42 91.1,50.47 C29.1 91.1,50.65 91.1,51.89 | 91.1,51.89 91.1,61.49 C66.1 91.1,61.67 89.85,62.92 | 91.1,51.89 v87.72,51.89 | 89.85,62.92 v88.79,62.92 | 78.83,18.47 78.83,26.29 79.9,27.36 79.9,27.89 C38.1 80.07,28.07 80.07,36.96 79.36,37.67 79.36,39.27 C21.1 79.36,39.45 v79.36,44.42 C50.1 79.36,50.65 79.36,61.49 C34.1 79.36,61.67 79.36,73.23 C57.1 79.36,73.41 79.36,78.03 | 78.83,18.47 78.83,17.22 C45.1 | 78.83,18.47 v77.76,18.47 | v89.32,44.42 91.1,44.42 | 87.72,6.55 90.39,6.55 C24.1 90.56,6.55 91.63,5.49 96.79,5.49 97.85,6.55 102.48,6.55 C46.1 102.65,6.73 102.65,17.04 C37.1 102.65,17.22 102.65,27.89 C39.1 102.48,28.07 101.23,29.31 | 87.72,6.55 83.1,6.55 82.03,5.49 79.9,5.49 78.83,6.55 C36.1 78.65,6.55 76.52,6.55 74.56,4.6 68.34,4.6 66.38,6.55 C35.1 | 87.72,6.55 87.72,7.98 | 87.72,7.98 v87.72,18.47 | 87.72,7.98 v88.79,7.98 | 101.23,29.31 v99.81,29.31 | 102.65,51.89 102.65,50.65 C51.1 102.65,50.47 102.65,39.45 C23.1 102.48,39.27 101.23,38.02 101.23,29.31 | 102.65,51.89 102.65,61.49 C67.1 102.48,61.67 101.23,62.92 | 102.65,51.89 v99.81,51.89 | 101.23,62.92 v99.63,62.92 | 102.48,75.13 102.48,84.96 C85.1 102.65,85.14 102.65,86.56 | 102.48,75.13 102.48,73.41 C59.1 102.48,73.23 101.23,71.98 101.23,62.92 | 102.65,86.56 102.65,96.16 C13.1 102.65,96.34 102.65,107.54 C27.1 102.48,107.72 101.23,108.97 v99.63,108.97 97.68,108.97 97.5,109.14 91.99,109.14 91.1,108.26
  Bottom 0.152: 102.65,86.56 v99.63,86.56 | 102.48,75.13 100.11,75.13 v99.63,74.65 | C12.1 91.1,96.34 91.1,107.54 C73.1 | 91.1,108.26 90.21,109.14 89.5,109.14 89.32,108.97 v87.72,108.97 83.99,108.97 83.81,109.14 80.43,109.14 79.36,108.08 | 91.1,108.26 91.1,107.72 C73.1 | 79.36,78.03 79.36,84.96 C83.1 79.36,85.14 79.36,96.16 C33.1 79.36,96.34 79.36,107.54 C72.1 | 79.36,78.03 v76.87,78.03 | 79.36,108.08 78.47,108.97 v75.98,108.97 67.63,108.97 66.38,107.72 C70.1 | 79.36,108.08 79.36,107.72 C72.1 | 79.36,108.08 C72.1 | 91.1,108.26 C73.1 | 66.38,51.89 66.38,50.83 66.56,50.65 C26.1 66.74,50.47 66.74,42.47 65.32,41.05 | 66.38,51.89 66.38,61.49 C64.1 66.38,61.67 66.38,73.23 C86.1 66.38,73.41 66.38,74.65 | 66.38,51.89 v64.6,51.89 | v63.54,40.69 64.25,40.69 64.6,41.05 65.32,41.05 | 65.32,41.05 66.21,40.16 66.21,39.45 C31.1 66.38,39.27 66.38,28.07 C16.1 66.21,27.89 v62.83,27.89 | 66.38,74.65 66.38,84.96 C80.1 66.38,85.14 66.38,86.56 | 66.38,86.56 v66.38,90.3 66.38,96.16 C76.1 66.38,96.34 v66.38,97.59 66.38,107.54 C70.1 | 66.38,74.65 v64.78,74.65 | 66.38,86.56 v64.6,86.56 | v63.54,108.97 64.96,108.97 66.21,107.72 C70.1 | 18.73,96.16 18.73,87.1 | 18.73,87.1 18.73,85.14 C11.1 | 18.73,96.16 24.96,96.16 | 24.96,96.16 28.51,96.16 C10.1 28.69,96.34 28.69,107.54 C53.1 | 18.73,96.16 C69.1 | 18.73,87.1 24.63,87.1 26.58,85.14 28.51,85.14 C75.1 28.69,84.96 28.69,73.41 C77.1 28.69,73.23 28.69,61.67 C82.1 28.69,61.49 28.69,50.65 C56.1 28.69,50.47 28.69,39.45 C61.1 28.51,39.27 28.51,38.2 | 24.96,96.16 v24.96,95.45 | C28.1 28.69,16.51 28.69,27.89 C48.1 28.51,28.07 28.51,33.05 27.8,33.76 27.8,36.78 28.51,37.49 28.51,38.2
  Bottom 0.152: C35.1 66.38,6.73 66.38,17.04 C68.1 | 54.29,8.33 54.29,6.73 C44.1 54.47,6.55 55.54,5.49 65.14,5.49 66.21,6.55 C35.1 | 54.29,8.33 54.29,11.71 53.4,12.6 53.4,16.69 C17.1 | 43.27,33.4 43.27,39.27 C52.1 | 43.27,33.4 43.27,28.07 C41.1 43.09,27.89 42.38,27.18 42.38,21.49 42.02,21.13 42.02,16.87 C22.1 41.23,16.15 41.23,8.83 42.55,7.52 C43.1 42.56,6.55 43.62,5.49 45.22,5.49 48.07,8.33 54.29,8.33 | 43.27,33.4 v42.56,33.4 | v40.96,40.69 41.85,40.69 43.09,39.45 C52.1 | 43.8,51.89 43.8,60.96 43.27,61.49 C62.1 43.09,61.67 42.02,62.74 v40.96,62.74 | 43.8,51.89 43.8,50.65 C25.1 | 43.8,51.89 v40.78,51.89 | 55,78.03 55,84.96 C79.1 | 55,78.03 55,73.41 C81.1 55,73.23 55,67.18 | 55,78.03 v52.51,78.03 | 55,55.27 55,61.49 C63.1 55,61.67 55,67.18 | 55,55.27 55,50.65 C47.1 54.83,50.47 54.83,49.4 | 55,55.27 v52.51,55.27 | 55,29.31 55,39.27 C30.1 54.83,39.45 53.58,40.69 | 55,29.31 55,28.07 C40.1 | 55,29.31 v51.45,29.31 | 53.58,40.69 v52.69,40.69 52.16,41.22 45.05,41.22 43.27,39.45 C52.1 | 54.83,49.4 54.83,41.94 53.58,40.69 | 54.83,49.4 44.87,49.4 44.69,49.58 44.69,49.76 43.98,50.47 C25.1 | 55,67.18 v55.04,67.18 | 28.51,38.2 31.53,38.2 C25.1
A0  (via drill 0.35)
  Top 0.152: v100.88,15.8 100.88,14.2 IC90.2 | v67.63,102.39 66.21,103.81 66.21,104.52 IC14.3
  Route3 0.152: v99.1,38.02 99.1,39.09 97.85,40.34 97.85,52.96 99.63,54.74 99.63,58.47 96.08,62.03 96.08,63.81 75.63,84.25 75.63,94.39 v67.63,102.39
  Bottom 0.152: v100.88,15.8 100.88,20.24 99.1,22.02 v99.1,38.02
A1  (via drill 0.35)
  Top 0.152: v69.05,102.39 68.87,102.39 67.45,103.81 67.45,104.52 IC14.4 | v76.52,17.93 76.52,17.22 77.05,16.69 77.05,14.2 IC93.2
  Bottom 0.152: v69.05,102.39 71.89,102.39 74.21,100.08 74.21,92.08 75.27,91.01 75.27,19.18 v76.52,17.93
A2  (via drill 0.35)
  Top 0.152: v78.83,1.4 77.23,3 77.23,3.53 IC96.2 | v74.92,109.68 72.43,109.68 71.72,108.97 69.76,108.97 68.69,110.03 68.69,110.57 IC14.10
  Bottom 0.152: v78.83,1.4 82.03,1.4 85.23,4.6 104.25,4.6 109.05,9.4 109.05,105.05 104.43,109.68 v74.92,109.68
A3  (via drill 0.35)
  Top 0.152: v98.21,5.84 90.56,5.84 88.96,4.24 88.96,3.71 IC99.2 | v77.05,108.26 69.23,108.26 67.45,110.03 67.45,110.57 IC14.11
  Route2 0.152: v98.21,5.84 98.21,6.73 110.12,18.64 110.12,90.12 98.03,102.21 98.03,103.45 93.94,107.54 77.76,107.54 v77.05,108.26
B0  (via drill 0.35)
  Top 0.152: v106.92,18.47 106.03,18.47 102.3,14.73 102.3,14.2 IC90.3 | IC18.3 102.23,102.65 101.97,102.39 101.97,102.33 v101.81,102.17
  Route2 0.152: v105.89,101.92 102.06,101.92 v101.81,102.17
  Bottom 0.152: v106.92,18.47 106.92,25.76 107.63,26.47 107.63,100.17 v105.89,101.92
B1  (via drill 0.35)
  Top 0.152: v79.72,18.47 78.47,17.22 78.47,14.2 IC93.3 | IC18.4 103.52,104.54 v103.52,103.22
  Route15 0.152: v79.72,18.47 79.72,22.02 97.85,40.16 97.85,52.96 98.21,53.31 98.21,73.94 98.92,74.65 98.92,97.98 103.52,102.58 v103.52,103.22
B2  (via drill 0.35)
  Top 0.152: v83.81,1.4 80.07,1.4 78.47,3 78.47,3.53 IC96.3 | v104.84,112.19 104.78,112.12 IC18.10
  Bottom 0.152: v83.81,1.4 91.45,1.4 91.63,1.22 101.94,1.22 109.77,9.04 109.77,105.41 104.84,110.34 v104.84,112.19
B3  (via drill 0.35)
  Top 0.152: v86.3,2.82 86.83,2.29 89.5,2.29 90.03,2.82 90.03,3.53 IC99.3 | v104.08,108.97 104.08,110.03 103.54,110.57 IC18.11
  Route2 0.152: v104.08,108.97 v108.71,108.97
  Bottom 0.152: v86.3,2.82 84.16,2.82 83.1,1.75 83.1,1.04 83.45,0.69 101.94,0.69 110.12,8.87 110.12,107.55 v108.71,108.97
C0  (via drill 0.35)
  Top 0.152: v106.39,17.58 103.54,14.73 103.54,14.2 IC90.4 | v67.45,94.74 67.09,94.74 66.21,93.85 66.21,93.14 IC23.3
  Route2 0.152: v106.39,17.58 106.39,17.93 106.21,18.11 106.21,23.44 109.41,26.65 109.41,79.63 98.03,91.01 98.03,92.08 93.94,96.16 71.89,96.16 69.76,94.03 68.16,94.03 v67.45,94.74
C1  (via drill 0.35)
  Top 0.152: v82.74,18.29 79.72,15.27 79.72,14.2 IC93.4 | v72.78,91.36 68.52,91.36 67.45,92.43 67.45,92.96 IC23.4
  Route3 0.152: v85.76,59 85.76,63.18 73.85,75.09 73.85,90.3 v72.78,91.36
  Bottom 0.152: v82.74,18.29 82.74,25.04 86.12,28.42 86.12,58.65 v85.76,59
C2  (via drill 0.35)
  Top 0.152: v81.67,7.98 79.72,6.02 79.72,3.71 IC96.4 | v71.89,101.32 69.58,101.32 68.69,100.43 68.69,99.37 IC23.10
  Route14 0.152: v85.41,17.04 74.92,27.53 74.92,38.38 v74.21,39.09
  Bottom 0.152: v81.67,7.98 81.67,13.31 v85.41,17.04 | v74.21,39.09 74.21,48.34 73.49,49.05 73.49,68.07 73.67,68.25 73.67,87.99 71.89,89.76 v71.89,101.32
C3  (via drill 0.35)
  Top 0.152: v91.99,1.93 91.45,2.46 91.45,3.53 IC99.4 | v64.96,101.68 66.03,101.68 67.27,100.43 67.27,99.37 IC23.11
  Bottom 0.152: v91.99,1.93 94.3,4.24 104.43,4.24 109.41,9.22 109.41,105.23 104.25,110.39 63.89,110.39 62.83,109.32 62.83,103.81 v64.96,101.68
D0  (via drill 0.35)
  Top 0.152: v107.63,17.76 104.79,14.91 104.79,14.2 IC90.5 | v101.94,90.65 101.94,92.79 102.12,92.96 IC28.3
  Route3 0.152: v107.63,17.76 107.63,30.91 106.21,32.33 106.21,70.21 103.9,72.52 103.9,85.32 101.94,87.27 v101.94,90.65
D1  (via drill 0.35)
  Top 0.152: IC93.5 80.96,15.44 v82.56,17.04 | v103.37,90.65 103.37,92.96 IC28.4
  Route14 0.152: v88.07,29.31 88.07,48.34 98.21,58.47 98.21,72.16 102.48,76.43 102.48,89.76 v103.37,90.65
  Bottom 0.152: v82.56,17.04 88.07,22.55 v88.07,29.31
D2  (via drill 0.35)
  Top 0.152: IC96.5 80.96,4.24 82.03,5.31 v82.92,5.31 | v105.14,97.59 104.96,97.59 104.78,97.77 IC28.10
  Route3 0.152: v82.92,5.31 83.63,5.31 84.34,4.6 103.9,4.6 108.34,9.04 108.34,30.73 107.63,31.45 107.63,95.1 v105.14,97.59
D3  (via drill 0.35)
  Top 0.152: v93.05,1.93 92.88,2.11 92.88,3.53 IC99.5 | v103.72,97.59 103.72,99.01 103.54,99.19 IC28.11
  Route2 0.152: v93.05,1.93 96.79,1.93 106.57,11.71 107.1,11.71 110.48,15.09 110.48,90.65 103.72,97.41 v103.72,97.59
E0  (via drill 0.35)
  Top 0.152: v105.5,21.84 106.03,21.31 106.03,20.24 IC90.9 | v65.67,79.1 65.67,81.59 66.03,81.94 IC33.3
  Route2 0.152: v105.5,45.31 104.97,45.31 97.32,52.96 96.08,52.96 83.45,65.58 78.3,65.58 77.41,66.47 77.41,68.96 69.05,77.32 67.27,77.32 66.38,78.21 66.38,78.38 v65.67,79.1
  Bottom 0.152: v105.5,21.84 105.5,28.6 106.03,29.13 106.03,44.78 v105.5,45.31
E1  (via drill 0.35)
  Top 0.152: v83.63,22.02 83.45,22.02 82.38,20.96 82.38,20.24 IC93.9 | v67.63,79.1 67.63,81.76 67.45,81.94 IC33.4
  Route3 0.152: v86.83,38.91 86.83,55.8 68.34,74.3 68.34,78.38 v67.63,79.1
  Bottom 0.152: v83.63,22.02 83.63,22.55 86.83,25.76 v86.83,38.91
E2  (via drill 0.35)
  Top 0.152: v82.38,11.35 82.38,9.75 IC96.9 | v67.63,86.56 68.52,87.45 68.52,88.16 IC33.10
  Route3 0.152: v69.76,84.25 67.63,86.39 v67.63,86.56
  Route14 0.152: v82.38,11.35 78.65,11.35 78.3,11 77.58,11 73.14,15.44 v73.14,23.98
  Bottom 0.152: v73.14,23.98 71.36,25.76 71.36,67.36 70.47,68.25 70.47,83.54 v69.76,84.25
E3  (via drill 0.35)
  Top 0.152: v94.3,11.35 94.12,11.18 94.12,9.75 IC99.9 | v74.56,83.54 74.56,86.56 71.18,89.94 68.52,89.94 67.45,88.88 67.45,88.16 IC33.11
  Route3 0.152: v98.92,55.45 98.92,57.94 91.84,65.01 85.28,65.01 74.56,75.73 v74.56,83.54
  Bottom 0.152: v94.3,11.35 94.3,17.4 98.74,21.84 98.74,36.07 97.32,37.49 97.32,40.51 101.41,44.6 101.59,44.6 101.94,44.96 101.94,48.69 98.92,51.71 v98.92,55.45
F0  (via drill 0.35)
  Top 0.152: v103.54,18.47 104.61,19.53 104.61,20.07 IC90.10 | v101.77,79.98 101.77,80 102.23,80.47 IC38.3
  Route3 0.152: v103.54,18.47 103.54,22.2 102.83,22.91 102.83,67.89 103.01,68.07 103.01,78.74 v101.77,79.98
F1  (via drill 0.35)
  Top 0.152: IC93.10 80.96,22.2 v82.03,23.27 | v103.19,80.34 103.37,80.34 103.5,80.42 IC38.4
  Route2 0.152: v88.79,78.56 89.85,78.56 90.03,78.74 101.59,78.74 v103.19,80.34
  Bottom 0.152: v82.03,23.27 82.03,24.87 84.7,27.53 84.7,74.47 v88.79,78.56
F2  (via drill 0.35)
  Top 0.152: v80.96,12.42 IC96.10 | v98.21,85.85 104.08,85.85 104.77,86.54 IC38.10
  Route15 0.152: v80.96,12.42 80.96,14.2 88.25,21.49 88.25,24.87 96.08,32.69 v96.08,34.65
  Bottom 0.152: v96.08,34.65 96.08,83.72 v98.21,85.85
F3  (via drill 0.35)
  Top 0.152: v98.56,9.58 97.32,8.33 93.59,8.33 92.88,9.04 92.88,9.58 IC99.10 | v103.72,86.56 103.72,87.99 103.54,88.16 IC38.11
  Route2 0.152: v98.56,9.58 100.52,9.58 109.77,18.82 109.77,80.52 v103.72,86.56
G0  (via drill 0.35)
  Top 0.152: v103.54,23.27 103.54,20.24 IC90.11 | v69.76,68.61 67.09,68.61 66.21,69.49 66.21,70.21 IC43.3
  Route2 0.152: v103.54,40.69 89.85,54.38 86.12,54.38 72.61,67.89 70.47,67.89 v69.76,68.61
  Route3 0.152: v103.54,40.69 v103.54,23.27
G1  (via drill 0.35)
  Top 0.152: v65.67,71.98 66.68,71.98 67.27,71.39 67.27,70.38 IC43.4 | v81.67,18.47 80.96,18.47 79.72,19.71 79.72,20.07 IC93.11
  Route14 0.152: v61.76,41.4 61.76,39.45 66.92,34.29 66.92,33.76 76.87,23.8 76.87,22.91 81.32,18.47 v81.67,18.47
  Bottom 0.152: v65.67,71.98 65.67,62.74 65.32,62.38 65.32,53.67 61.76,50.11 v61.76,41.4
G2  (via drill 0.35)
  Top 0.152: v78.65,12.42 79.54,11.53 79.54,9.75 IC96.11 | v71.01,84.07 70.65,84.07 69.94,83.36 69.41,83.36 69.23,83.19 69.23,80.16 68.69,79.63 68.69,76.43 IC43.10
  Route14 0.152: v78.65,12.42 73.85,17.22 73.85,24.33 v73.14,25.04
  Bottom 0.152: v73.14,25.04 73.14,36.07 72.61,36.6 72.61,66.47 72.96,66.83 72.96,67.54 71.89,68.61 71.89,82.47 71.01,83.36 v71.01,84.07
G3  (via drill 0.35)
  Top 0.152: v91.45,7.98 91.45,9.58 IC99.11 | v67.63,78.03 67.63,76.61 67.45,76.43 IC43.11
  Route2 0.152: v85.59,72.34 83.1,72.34 82.8,72.64 82.66,72.64 74.26,72.64 68.87,78.03 v67.63,78.03
  Bottom 0.152: v91.45,7.98 91.45,14.38 89.5,16.33 89.5,21.31 89.67,21.49 89.67,37.67 86.47,40.87 86.47,60.43 85.59,61.32 v85.59,72.34
GND  (via drill 0.35)
  Top 0.152: 80.96,31.62 IC85.12 | 80.96,31.62 81.67,32.33 83.99,32.33 84.7,31.62 84.7,31.09 IC85.9 | 72.25,32.33 72.25,35.18 71.18,36.25 IC73.7 | 72.25,32.33 72.25,29.67 71.18,28.6 71.18,24.87 IC83.7 | 80.96,31.62 80.25,32.33 76.52,32.33 | 72.25,32.33 76.52,32.33 | IC86.7 IC86.8 96.61,24.87 96.61,30.91 IC86.9 96.43,31.09 96.43,31.62 95.72,32.33 93.41,32.33 | 80.61,26.29 81.5,27.18 82.74,27.18 83.45,26.47 83.45,24.87 IC85.7 84.7,24.87 | 80.61,26.29 79.72,25.4 79.72,24.87 IC85.4 | 91.45,27.36 91.45,29.13 92.7,30.38 92.7,30.91 IC86.12 92.88,31.09 92.88,31.8 93.41,32.33 | 91.45,27.36 IC86.4 | 91.45,27.36 88.25,27.36 85.76,24.87 IC85.8 84.7,24.87 | 107.45,6.02 107.45,7.98 107.99,8.51 107.99,13.49 107.45,14.02 IC90.7 107.45,14.2 108.34,15.09 108.34,20.96 107.45,21.84 107.45,24.87 IC88.7 | 107.45,6.02 107.45,3.71 IC100.7 | 86.65,17.22 93.23,17.22 95.19,15.27 95.19,14.2 IC91.7 | 86.65,17.22 IC93.7 83.63,14.02 84.16,13.49 84.16,8.51 83.63,7.98 83.63,3.71 IC96.7 83.63,3.53 85.94,1.22 93.41,1.22 95.19,3 95.19,3.53 IC99.7 95.36,3.71 97.14,3.71 99.45,6.02 107.45,6.02 | 84.7,24.87 84.7,19.18 86.65,17.22 | 76.52,32.33 76.52,28.96 77.58,27.89 79.01,27.89 80.61,26.29 | IC14.7 71.18,104.7 73.67,104.7 75.98,107.01 78.65,107.01 79.54,106.12 79.54,104.7 IC12.4 79.72,104.52 79.72,103.99 80.61,103.1 82.56,103.1 83.45,103.99 83.45,104.52 IC12.7 | 92.88,106.48 93.41,107.01 94.48,107.01 95.19,106.3 95.19,104.7 IC16.7 95.36,104.7 96.43,104.7 IC16.8 | 92.88,106.48 91.45,105.05 91.45,104.7 IC16.4 91.27,104.52 91.27,103.81 90.56,103.1 86.3,103.1 84.87,104.52 IC12.8 84.7,104.7 83.63,104.7 IC12.7
  Top 0.152: IC16.9 96.43,110.57 96.43,110.03 95.72,109.32 93.59,109.32 92.88,110.03 92.88,110.57 IC16.12 92.7,110.74 92.7,111.28 91.81,112.17 86.3,112.17 84.87,110.74 IC12.9 84.7,110.57 84.7,108.61 82.92,106.83 | IC12.12 80.96,108.79 82.92,106.83 | 82.92,106.83 83.45,106.3 83.45,104.7 IC12.7 | 93.41,77.67 93.59,77.85 95.72,77.85 96.43,77.14 96.43,76.43 IC46.9 | 93.41,77.67 92.88,77.14 92.88,76.43 IC46.12 | IC36.8 96.43,82.12 95.36,82.12 IC36.7 95.19,81.94 95.19,81.41 v94.12,80.34 | v93.05,78.03 93.41,77.67 | v93.05,106.3 92.88,106.48 | v93.05,32.69 93.41,32.33 | IC66.12 92.88,53.67 92.88,54.2 93.94,55.27 95.9,55.27 96.43,54.74 96.43,53.67 IC66.9 96.61,53.49 97.07,53.49 v97.55,53.98 | IC56.7 95.36,58.65 96.43,58.65 IC56.8 96.61,58.47 97.32,58.47 98.92,56.87 v101.6,56.87 v104.43,56.87 107.99,56.87 | 107.99,56.87 107.99,57.94 107.45,58.47 IC58.7 | 107.99,56.87 107.99,52.43 107.45,51.89 107.45,47.45 IC68.7 | 107.45,73.05 107.45,74.65 107.99,75.18 107.99,79.98 107.31,80.65 IC38.7 107.31,83.57 107.99,84.24 107.99,89.41 107.45,89.94 107.45,92.96 IC28.7 107.45,93.14 107.99,93.68 107.99,100.43 107.45,100.97 107.45,104.52 IC18.7 | 107.45,73.05 107.45,70.38 IC48.7 | 91.45,69.67 91.45,70.21 IC46.4 91.45,69.67 | 91.45,69.67 92.16,68.96 94.48,68.96 95.19,69.67 95.19,70.21 IC46.7 95.36,70.38 96.43,70.38 IC46.8 96.52,72.26 97.31,73.05 105.85,73.05 | 91.45,69.67 90.74,68.96 86.12,68.96 84.87,70.21 IC45.8 84.87,70.38 84.87,76.25 IC45.9 84.7,76.43 84.7,77.14 83.99,77.85 81.85,77.85 80.96,76.96 | IC45.4 79.72,70.21 79.72,69.67 80.43,68.96 82.74,68.96 83.45,69.67 83.45,70.21 IC45.7 83.45,70.38 83.45,71.98 80.25,75.18
  Top 0.152: 80.25,75.18 80.96,75.89 IC45.12 80.96,76.96 | 80.25,75.18 78.65,73.58 75.81,73.58 72.61,70.38 71.18,70.38 IC43.7 | 92.88,87.45 92.88,88.16 IC36.12 92.88,87.45 | 92.88,87.45 94.48,85.85 95.72,85.85 96.43,86.56 96.43,88.16 IC36.9 | 83.63,82.12 84.7,82.12 IC35.8 84.87,81.94 85.23,81.59 | 85.23,81.59 86.12,80.7 88.07,80.7 88.25,80.87 88.25,83.19 88.43,83.36 90.74,83.36 91.27,82.83 91.27,82.12 IC36.4 | 92.88,87.45 92.52,87.45 90.56,85.5 89.14,85.5 85.23,81.59 | IC41.12 56.6,76.43 56.6,77.14 57.32,77.85 59.45,77.85 60.16,77.14 60.16,76.43 IC41.9 60.34,76.25 61.76,76.25 64.07,73.94 67.98,73.94 69.23,75.18 69.23,79.63 71.01,81.41 71.01,81.94 IC33.7 71.18,82.12 74.03,82.12 | 74.03,82.12 74.21,82.12 75.45,83.36 78.83,83.36 | 78.83,83.36 79.54,82.65 79.54,82.12 IC35.4 | 80.96,85.85 80.96,85.5 78.83,83.36 | 80.96,85.85 v80.96,86.56 IC35.12 | 80.96,85.85 83.63,85.85 | 83.63,85.85 83.99,85.85 84.7,86.56 84.7,88.16 IC35.9 | 83.63,85.85 83.63,82.12 | 83.63,82.12 IC35.7 | 80.96,76.96 79.01,78.92 77.23,78.92 74.03,82.12 | 105.85,73.05 107.45,73.05 | 78.47,94.56 78.83,94.56 79.54,93.85 79.54,93.14 IC25.4 | 78.47,94.56 75.45,94.56 74.03,93.14 71.18,93.14 IC23.7 | 78.47,94.56 80.96,97.05 v80.96,97.59 IC25.12 80.96,100.69 81.04,100.77 84.46,100.77 84.7,100.53 84.7,99.37 IC25.9 84.7,99.19 84.7,96.16 | 91.45,93.02 91.45,92.96 91.45,92.61 IC26.4 91.45,93.02 | IC26.8 96.43,93.14 95.36,93.14 IC26.7 95.19,92.96 95.19,91.8 94.32,90.93 91.97,90.93 91.45,91.44 91.45,91.72 91.44,91.72 | IC26.9 96.43,99.37 96.43,99.9 95.72,100.61 93.41,100.61 92.88,100.08 92.88,99.37 IC26.12 92.7,99.19 92.7,97.7 91.16,96.16 84.7,96.16
  Top 0.152: 84.7,93.14 83.63,93.14 IC25.7 | 84.7,93.14 84.7,96.16 | 84.7,93.14 IC25.8 84.87,92.96 86.12,91.72 91.44,91.72 | IC78.7 107.28,36.42 107.28,36.96 105.5,38.73 97.85,38.73 96.61,37.49 96.61,36.42 IC76.8 96.43,36.42 95.36,36.42 IC76.7 95.19,36.42 95.19,37.75 94.2,38.73 91.81,38.73 91.45,38.38 91.45,36.42 IC76.4 91.43,35.06 91.06,34.68 86.44,34.68 84.87,36.25 IC75.8 | 92.88,41.76 92.88,42.29 IC76.12 92.88,41.76 | 92.88,41.76 94.83,39.8 95.72,39.8 96.43,40.51 96.43,42.29 IC76.9 | IC75.12 80.96,43.8 81.24,44.07 v81.32,44.07 81.34,44.05 84.28,44.05 84.7,43.64 84.7,42.47 IC75.9 84.87,42.29 84.87,39.62 | IC75.4 79.72,36.25 79.72,35.71 80.43,35 82.74,35 83.45,35.71 83.45,36.25 IC75.7 83.63,36.42 84.7,36.42 IC75.8 | 84.87,39.62 84.87,36.42 IC75.8 | 92.88,41.76 92.52,41.76 90.39,39.62 84.87,39.62 | 105.85,73.05 v105.85,73.23 | v34.02,60.25 34.02,58.65 IC113.8 | 33.85,107.37 33.85,107.39 32.09,109.14 | 33.85,107.37 33.85,104.7 IC117.8 | 32.09,109.14 31.53,109.7 31.53,110.57 IC117.11 | 33.85,107.37 41.31,107.37 43.45,105.23 43.45,104.7 IC10.4 | 14.41,102.21 11.74,104.88 IC9.8 11.09,104.88 11.09,106.22 8.6,108.71 8.6,110.92 IC9.11 | IC15.7 13.93,99.37 13.93,101.76 14.38,102.21 14.41,102.21 | 27.62,112.17 IC117.14 | 27.62,112.17 30.65,115.19 GND.1 | 21.58,104.7 20.33,104.7 IC34.6 20.15,104.7 19.09,104.7 IC34.5 18.91,104.52 18.91,102.7 18.42,102.21 14.41,102.21 | IC34.8 21.58,110.74 20.33,110.74 IC34.9 20.15,110.74 20.15,111.45 19.44,112.17 16.6,112.17 | 16.6,112.17 16.6,110.74 IC34.12 | 21.58,104.7 21.58,110.57 IC34.8 | 21.58,104.7 IC34.7 | 27.62,112.17 21.91,112.17 21.59,111.85 IC34.8
  Top 0.152: v32.07,109.14 32.09,109.14 | IC8.7 9.84,13.67 10.49,13.67 13.99,10.17 19.92,10.17 21.58,11.82 21.58,13.31 IC32.7 21.76,13.49 v21.76,15.44 21.76,15.5 22.29,16.03 22.29,22.27 21.6,22.96 IC29.7 | IC1.7 9.84,92.25 12.03,90.07 12.03,88.11 | IC4.7 9.84,40.34 10.91,41.4 10.91,44.78 | 10.91,44.78 10.91,46.91 9.84,47.98 IC2.7 | 23.18,44.6 23.18,44.74 21.59,46.32 IC24.7 21.59,49.03 22.61,50.04 22.61,56.17 21.6,57.17 IC17.7 21.59,60.27 23.71,62.39 23.71,70.03 23.36,70.38 23.08,70.38 | 23.18,44.6 23.18,37.85 21.76,36.42 IC27.7 21.76,36.25 22.64,35.36 22.64,25.29 22.23,24.87 IC29.7 | 23.08,70.38 21.76,70.38 IC13.7 | 10.91,44.78 18.91,44.78 19.09,44.6 23.18,44.6 | 23.08,70.38 23.08,77.81 21.8,79.1 12.51,79.1 9.84,81.76 IC3.7 9.84,83.9 12.03,86.08 12.03,88.11 | IC29.7 | v4.69,109.64 4.69,110.92 IC9.14 | v9.84,62.33 9.84,63.81 10.55,64.52 10.55,70.03 9.84,70.74 IC5.7 | v9.84,62.33 IC7.7 | IC6.7 9.84,26.62 v9.89,26.66 | v9.85,62.33 v9.84,62.33 | 58.92,1.58 58.56,1.22 51.8,1.22 49.49,3.53 47.36,3.53 IC98.7 | 58.92,1.58 58.92,3.53 IC92.7 | 58.92,1.58 58.92,1.45 69.46,1.45 71.01,3 71.01,3.53 IC97.7 71.18,3.71 v71.18,5.31 | v72.07,15.27 72.07,15.09 71.18,14.2 IC94.7 | 34.73,46.56 34.73,39.27 34.02,38.56 34.02,36.42 IC111.8 34.02,36.25 34.02,34.11 35.8,32.33 39,32.33 | 34.73,46.56 34.02,47.27 IC112.8 | 47.71,54.92 45.58,54.92 44.87,54.2 44.87,53.67 IC60.12 | 47.71,54.92 48.43,54.2 48.43,53.67 IC60.9 48.6,53.49 48.6,47.45 IC60.8 48.43,47.45 47.36,47.45 IC60.7 47.18,47.27 47.18,46.74 46.47,46.03 44.34,46.03 43.62,46.74 43.62,47.27 IC60.4 43.45,47.45 43.45,47.98 42.2,49.23 39.18,49.23 36.51,46.56 34.73,46.56
  Top 0.152: IC50.4 43.62,58.65 43.62,59.18 44.34,59.89 46.47,59.89 47.18,59.18 47.18,58.65 IC50.7 47.36,58.65 48.43,58.65 IC50.8 48.43,58.47 48.43,56.69 | 47.71,54.92 47.71,55.98 48.43,56.69 | 60.16,24.87 60.16,19.18 59.09,18.11 59.09,13.84 IC22.8 | 60.16,24.87 IC81.7 | 60.16,24.87 IC81.8 60.34,24.87 60.34,30.91 IC81.9 60.16,31.09 60.16,32.69 59.45,33.4 58.38,33.4 56.6,31.62 56.6,31.09 IC81.12 56.43,30.91 56.43,30.38 55.36,29.31 55.36,24.87 IC81.4 55.18,24.87 55.18,24.16 53.76,22.73 48.78,22.73 | 48.78,22.73 48.78,24.69 48.6,24.87 IC80.8 47.36,24.87 | 48.78,22.73 48.78,18.47 47.36,17.04 47.36,13.84 IC108.8 | 34.2,24.69 34.02,24.87 IC110.8 34.2,24.69 | 34.2,24.69 34.73,24.16 34.73,18.47 34.02,17.76 34.02,13.49 IC109.8 | 43.62,38.73 43.62,40.16 44.69,41.22 44.69,42.29 IC70.12 | 43.62,38.73 43.62,36.42 IC70.4 43.45,36.25 43.45,35.24 42.22,34.01 40.68,34.01 39,32.33 | IC70.7 47.36,36.42 48.43,36.42 IC70.8 | 48.6,38.2 48.6,36.42 IC70.8 | 48.6,38.2 48.6,42.29 IC70.9 | 43.62,38.73 46.47,38.73 47,38.2 48.6,38.2 | 55.36,35.53 55.36,36.25 IC71.4 55.36,35.53 | 55.36,35.53 55.89,35 58.38,35 58.92,35.53 58.92,36.25 IC71.7 59.09,36.42 60.16,36.42 IC71.8 | 44.69,29.67 44.69,30.91 IC80.12 | 44.69,29.67 44.69,29.13 43.62,28.07 43.62,24.87 IC80.4 | 44.69,29.67 47.36,29.67 | 47.36,29.67 47.71,29.67 48.43,30.38 48.43,30.91 IC80.9 48.6,31.09 49.85,32.33 | 55.36,35.53 55,35.53 51.8,32.33 49.85,32.33 | 49.85,32.33 48.6,33.58 48.6,36.25 IC70.8 | 34.2,24.69 39,29.49 39,32.33 | 47.36,29.67 47.36,24.87 | 47.36,24.87 IC80.7 | 92.88,63.98 92.88,64.52 IC56.12 92.88,63.98 | 92.88,63.98 94.65,62.2 95.72,62.2 96.43,62.92 96.43,64.52 IC56.9
  Top 0.152: IC55.12 80.96,65.23 81.85,66.12 83.81,66.12 84.7,65.23 84.7,64.69 IC55.9 84.87,64.52 84.87,61.85 | 79.72,57.94 79.72,58.47 IC55.4 79.72,57.94 | 79.72,57.94 80.43,57.23 82.74,57.23 83.45,57.94 83.45,58.47 IC55.7 83.63,58.65 84.7,58.65 IC55.8 | IC56.4 91.27,58.47 91.27,57.76 90.39,56.87 86.47,56.87 84.87,58.47 IC55.8 | 84.87,61.85 84.87,58.65 IC55.8 | 92.88,63.98 92.52,63.98 90.39,61.85 84.87,61.85 | 91.45,46.91 91.45,47.27 IC66.4 91.45,46.91 | 91.45,46.91 92.34,46.03 94.48,46.03 95.19,46.74 95.19,47.27 IC66.7 95.36,47.45 96.43,47.45 IC66.8 | 80.96,54.2 IC65.12 | 80.96,54.2 81.67,54.92 83.99,54.92 84.7,54.2 84.7,53.67 IC65.9 84.7,53.49 84.7,47.45 | 84.7,47.45 83.63,47.45 IC65.7 83.45,47.27 83.45,46.74 82.74,46.03 80.43,46.03 79.72,46.74 79.72,47.27 IC65.4 79.54,47.45 79.54,48.16 78.12,49.58 77.05,49.58 71.18,55.45 71.18,55.98 | 84.7,47.45 IC65.8 84.87,47.27 86.47,45.67 90.21,45.67 91.45,46.91 | 79.72,57.94 76.52,54.74 76.52,52.43 76.7,52.25 77.76,52.25 77.76,54.74 77.94,54.92 80.25,54.92 80.96,54.2 | IC115.8 34.02,81.94 34.02,80.16 34.38,79.81 41.85,79.81 43.45,81.41 43.45,81.94 IC30.4 43.62,82.12 43.62,85.14 44.69,86.21 44.69,88.16 IC30.12 44.87,88.16 44.87,88.88 45.58,89.59 47.71,89.59 48.43,88.88 48.43,88.16 IC30.9 48.6,88.16 48.6,85.85 | 57.14,83.36 58.2,83.36 58.92,82.65 58.92,82.12 IC31.7 59.09,82.12 60.16,82.12 IC31.8 | 57.14,83.36 56.07,83.36 55.36,82.65 55.36,82.12 IC31.4 55.18,81.94 55.18,81.41 54.47,80.7 49.85,80.7 48.6,81.94 IC30.8 | IC31.9 60.16,88.16 60.16,88.88 59.45,89.59 57.32,89.59 56.6,88.88 56.6,88.16 IC31.12 56.43,88.16 56.43,87.45 54.83,85.85 48.6,85.85
  Top 0.152: IC30.7 47.36,82.12 48.43,82.12 IC30.8 | 48.6,85.85 48.6,82.12 IC30.8 | 55.36,57.76 55.36,58.47 IC51.4 55.36,57.76 | 55.36,57.76 55.89,57.23 58.38,57.23 58.92,57.76 58.92,58.47 IC51.7 59.09,58.65 60.16,58.65 | 60.16,58.65 60.16,60.96 60.52,61.32 68.87,61.32 71.01,59.18 71.01,58.65 IC53.7 71.18,58.47 71.18,55.98 | 60.16,58.65 IC51.8 | IC114.8 34.02,70.21 36.33,70.21 37.93,68.61 42.38,68.61 43.45,69.67 43.45,70.21 IC40.4 43.62,70.38 43.62,70.92 44.69,71.98 44.69,76.25 IC40.12 44.87,76.43 44.87,77.67 45.62,78.42 47.14,78.42 48.43,77.14 | 55.36,69.67 55.36,70.21 IC41.4 55.36,69.67 | 55.36,69.67 56.07,68.96 58.38,68.96 58.92,69.49 58.92,70.21 IC41.7 59.09,70.38 60.16,70.38 IC41.8 | 57.32,63.27 58.38,62.2 59.98,62.2 60.34,62.56 60.34,64.52 IC51.9 | 57.32,63.27 56.6,63.98 56.6,64.52 IC51.12 | 47.18,66.12 47.71,66.12 48.43,65.41 48.43,64.69 IC50.9 48.6,64.52 50.74,62.38 | 47.18,66.12 45.58,66.12 44.87,65.41 44.87,64.69 IC50.12 | IC40.8 48.43,70.38 47.36,70.38 IC40.7 47.18,70.21 47.18,66.12 | IC40.9 48.6,76.25 48.6,75.25 49.37,74.48 49.37,72.21 48.6,71.44 48.6,70.38 IC40.8 | 57.32,63.27 56.25,62.2 50.91,62.2 50.74,62.38 | 55.36,69.67 54.29,68.61 50.2,68.61 48.6,70.21 IC40.8 | 48.43,77.14 48.43,76.43 IC40.9 | 55.36,57.76 55,57.76 54.47,57.23 50.91,57.23 50.74,57.4 50.74,62.38 | 57.14,83.36 57.14,80.87 55,78.74 50.03,78.74 48.43,77.14 | 48.43,77.14 IC40.9 | 48.43,56.69 50.38,56.69 51.09,55.98 v56.78,55.98 71.18,55.98 | 55.18,106.48 55.18,104.7 IC11.4 | 55.18,106.48 55.54,106.83 57.32,106.83 58.92,105.23 58.92,104.7 IC11.7 | IC11.8 60.16,104.7 59.09,104.7 IC11.7
  Top 0.152: IC10.7 47.36,104.7 48.43,104.7 IC10.8 48.6,104.7 48.6,107.01 | IC10.12 44.87,110.74 44.87,111.99 45.4,112.52 47.99,112.52 48.43,112.09 48.43,110.74 IC10.9 48.6,110.57 48.6,107.01 | 55.18,106.48 54.83,106.48 54.29,107.01 48.6,107.01 | 56.43,94.92 56.96,95.45 58.2,95.45 58.92,94.74 58.92,93.14 IC21.7 | 56.43,94.92 55.36,93.85 55.36,93.14 IC21.4 | IC21.8 60.16,93.14 59.09,93.14 IC21.7 | 48.43,100.97 47.71,101.68 46.65,101.68 44.87,99.9 44.87,99.37 IC20.12 | 48.43,100.97 48.43,99.37 IC20.9 48.43,99.19 48.43,98.3 45.58,95.45 | 45.58,95.45 47.18,93.85 47.18,93.14 IC20.7 | 45.58,95.45 45.05,95.99 38.25,95.99 35.4,93.14 34.02,93.14 IC116.8 | IC20.7 47.18,92.96 47.18,91.48 46.67,90.96 44.29,90.96 43.5,91.76 IC20.4 | IC20.7 47.36,93.14 48.43,93.14 IC20.8 48.6,92.96 48.6,91.9 49.14,91.36 57.85,91.36 58.92,92.43 58.92,92.96 IC21.7 | 48.43,100.97 49.85,102.39 57.49,102.39 58.92,103.81 58.92,104.52 IC11.7 | 56.66,109.02 56.68,109 59.13,109 60.16,110.03 60.16,110.57 IC11.9 | 56.66,109.02 56.6,109.08 56.6,110.57 IC11.12 | 57.32,100.61 56.6,99.9 56.6,99.37 IC21.12 | 57.32,100.61 59.63,100.61 60.16,100.08 60.16,99.37 IC21.9 | v56.96,100.97 57.32,100.61 | v56.6,108.97 56.66,109.02 | v56.6,94.74 56.43,94.92 | 56.6,49.4 56.96,49.76 58.38,49.76 58.92,49.23 58.92,47.45 IC61.7 59.09,47.45 60.16,47.45 IC61.8 60.34,47.45 63,50.11 67.98,50.11 69.23,48.87 69.23,46.2 69.41,46.03 70.29,46.03 71.01,46.74 71.01,47.27 IC63.7 | 56.6,49.4 55.36,48.16 55.36,47.45 IC61.4 | IC61.9 60.16,53.67 60.16,54.2 59.45,54.92 57.32,54.92 56.6,54.2 56.6,53.67 IC61.12 56.6,53.49 v56.6,51.89 | 57.32,41.05 56.6,41.76 56.6,42.29 IC71.12
  Top 0.152: 57.32,41.05 59.45,41.05 60.16,41.76 60.16,42.29 IC71.9 | v57.14,40.87 57.32,41.05 | v56.96,49.05 56.6,49.4 | 16.6,112.17 15.72,112.17 15.24,111.69 IC34.13 | IC19.7 12.03,88.1 12.03,88.11 | 91.44,91.72 91.45,91.73 91.45,93.02
  Route2 0.152: v101.6,56.87 98.7,53.98 v97.55,53.98
  Bottom 0.152: C24.2 92.34,6.73 92.34,17.04 C42.2 92.52,17.22 93.05,17.76 93.05,27.89 C15.2 93.05,28.07 v93.05,32.69 93.05,39.62 C20.2 93.05,39.8 93.05,50.47 C29.2 93.05,50.65 93.05,61.49 C66.2 93.05,61.67 93.05,71.13 93.32,71.39 93.32,71.94 93.05,72.2 93.05,73.23 C58.2 93.05,73.41 v93.05,78.03 93.05,80.34 | 93.05,80.34 93.05,84.96 C84.2 93.05,85.14 93.05,90.49 93.66,91.1 93.66,92.89 93.05,93.5 93.05,93.68 | 93.05,93.68 93.05,96.16 C12.2 93.05,96.34 v93.05,106.3 93.05,107.54 C73.2 | 93.05,80.34 v94.12,80.34 | C27.2 104.43,107.54 104.43,96.34 C13.2 104.43,96.16 104.43,85.14 C85.2 104.43,84.96 104.43,78.56 104.25,78.38 104.25,73.58 104.43,73.41 C59.2 | C46.2 104.43,6.73 104.43,17.04 C37.2 104.43,17.22 104.43,27.89 C39.2 104.43,28.07 104.43,39.27 C23.2 104.43,39.45 104.43,50.47 C51.2 104.43,50.65 v104.43,56.87 104.43,61.49 C67.2 104.43,61.67 104.43,73.23 C59.2 | 81.32,86.56 81.32,85.14 C83.2 81.32,84.96 81.32,73.41 C57.2 81.32,73.23 81.32,61.67 C34.2 81.32,61.49 81.32,50.65 C50.2 81.32,50.47 v81.32,44.07 81.32,39.45 C21.2 81.32,39.27 81.85,38.73 81.85,28.07 C38.2 81.85,27.89 80.78,26.82 80.78,17.22 C45.2 80.61,17.04 80.61,15.44 75.63,10.47 75.63,7.62 76.34,6.91 | 81.32,86.56 81.32,95.45 | 81.32,95.45 81.32,96.16 C33.2 | 81.32,97.59 81.32,96.34 C33.2 | 81.32,97.59 81.32,107.54 C72.2 | 81.32,97.59 v80.96,97.59 | 81.32,86.56 v80.96,86.56 | v105.85,73.23 104.61,73.23 C59.2 | 93.05,93.68 85.41,93.68 83.63,95.45 81.32,95.45 | 81.32,95.45 C33.2 | C25.2 45.58,50.65 45.58,61.14 45.22,61.49 C62.2 45.05,61.67 43.27,63.45 | C61.2 30.47,39.45 30.47,50.47 C56.2 30.47,50.65 30.47,60.25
